(* Logix 5000 AddOnInstructionDefinition export Banner_R95C_4B4UI_Param_v4; software revision 36.00 *)

TYPE Banner_Direct1_v4 :
STRUCT
   Reserved : INT;
   Master_Cycle_Time : INT;
   Min_Cycle_Time : INT;
   M_Sequence_Capability : INT;
   IO_Link_Version_ID : INT;
   Process_Data_Input_Length : INT;
   Process_Data_Output_Length : INT;
   Vendor_ID1 : INT;
   Vendor_ID2 : INT;
   Device_ID1 : INT;
   Device_ID2 : INT;
   Device_ID3 : INT;
END_STRUCT
END_TYPE

TYPE Banner_IOL_Port_v4 :   // UDT that has all of the data items necessary to communicate with a specific Port on a IO-Link Master
STRUCT
   Port_Controlled : INT;   // Each bit represents a port on an IO-Link Master. Set to 1 to tell AOI to control that port.
   Port_Activate : INT;   // Each bit represents a port on an IO-Link Master. When ON that port will process any commands in queue.
   Port_Read : INT;   // Each bit represents a port on an IO-Link Master. Used to determine when device AOI has requested a Read command.
   Port_Write : INT;   // Each bit represents a port on an IO-Link Master. Used to determine when device AOI has requested a Write command.
   Port_RW_Complete : INT;   // Each bit represents a port on an IO-Link Master. Tells device AOI that Read or Write request has been completed.
   Port_Device_Read : INT;
   Data_Transfer : SINT[190];   // Array to transfer data from IO-Master to device AOIs.
END_STRUCT
END_TYPE

TYPE Banner_Locks_v4 :
STRUCT
   Parameter_Access_Lock : SINT;   // Write access to all parameters is prohibited while value is 1. Only this parameter can be adjusted when value is 1.
   Data_Storage_Lock : SINT;   // Automatic data storage is disabled when this value is equal to 1. Read access is not affected.
   Local_Parameterization_Lock : SINT;   // Parameterization via local control elements on device is disabled.
   Local_User_Interface_Lock : SINT;   // Operation of local user interface is disabled.
END_STRUCT
END_TYPE

TYPE Banner_R95C_4B4UI_IO_Metrics_v4 :
STRUCT
   Port_Discrete2_Totalizer : DINT;
   Port_Discrete2_Events_Per_Minute : DINT;
   Port_Discrete2_Duration : DINT;
   Port_Discrete2_Count : DINT;
   Port_Discrete1_Totalizer : DINT;
   Port_Discrete1_Events_Per_Minute : DINT;
   Port_Discrete1_Duration : DINT;
   Port_Discrete1_Count : DINT;
END_STRUCT
END_TYPE

TYPE Banner_R95C_4B4UI_MDC_v4 :   // MDC Descriptor parameters for Smart Sensor Profile 2nd edition.
STRUCT
   Lower_Limit : DINT;
   Upper_Limit : DINT;
   Unit : INT;   // 1209 = A, 1240 = V
   Scale : SINT;
END_STRUCT
END_TYPE

TYPE Banner_R95C_4B4UI_Metrics_v4 :
STRUCT
   Port4 : Banner_R95C_4B4UI_IO_Metrics_v4;
   Port3 : Banner_R95C_4B4UI_IO_Metrics_v4;
   Port2 : Banner_R95C_4B4UI_IO_Metrics_v4;
   Port1 : Banner_R95C_4B4UI_IO_Metrics_v4;
END_STRUCT
END_TYPE

TYPE Banner_R95C_4B4UI_Port_Config_v4 :
STRUCT
   D2 : Banner_R95C_4B4UI_Port_Discrete_v4;   // Discrete 2
   D1 : Banner_R95C_4B4UI_Port_Discrete_v4;   // Discrete 1
END_STRUCT
END_TYPE

TYPE Banner_R95C_4B4UI_Port_Discrete_v4 :
STRUCT
   PFM_Far_Freq : DINT;   // 100 to 600.
   PFM_Near_Freq : DINT;   // 100 to 600.
   Mirroring_Inversion : SINT;   // 0 = Not Inverted, 1 = Inverted.
   Mirroring_Channel_Selection : SINT;   // 0 = Discrete 1, 1 = Discrete 2.
   Mirroring_Port_Selection : SINT;   // 0 = Port1, 1 = Port2, 2 = Port3, 3 = Prot4, 4 = Prot5, 5 = Port6, 6 = Port7, 7 = Port8.
   Mirroring_Enable : SINT;   // 0 = Disabled, 1 = Enabled.
   Delay_Timer2 : DINT;
   Delay_Timer1 : DINT;
   Delay_Mode : SINT;   // 0=Disabled,1=On Off Delay, 2=On OneShot, 3=Off OneShot, 4=On Pulse Stretcher, 5=Off Pulse Stretcher, 6=Totalizer, 7=Retriggerable On OneShot, 8=Retriggerable Off OneShot.
   IO : SINT;   // 0=NPN, 1=PNP
END_STRUCT
END_TYPE

TYPE Banner_R95C_4B4UI_Port_Mirroring_v4 :
STRUCT
   Output_Enable : SINT;   // 0 = Disabled, 1 = Enabled. Enable mirroring over output analog channel.
   Port_Selection : SINT;   // 0 = Port 5, 1 = Port 6, 2 = Port 7, 3 = Port 8. Input port to mirror over output analog channel.
END_STRUCT
END_TYPE

TYPE Banner_R95C_4B4UI_POVR1_v4 :
STRUCT
   PDO8_OVD : SINT;   // 0 = Hold, 1 = Low, 2 = High. Value sensor will output when PDO value is not within allowable range.
   PDO7_OVD : SINT;   // 0 = Hold, 1 = Low, 2 = High. Value sensor will output when PDO value is not within allowable range.
   PDO6_OVD : SINT;   // 0 = Hold, 1 = Low, 2 = High. Value sensor will output when PDO value is not within allowable range.
   PDO5_OVD : SINT;   // 0 = Hold, 1 = Low, 2 = High. Value sensor will output when PDO value is not within allowable range.
END_STRUCT
END_TYPE

TYPE Banner_R95C_4B4UI_RD_v4 :   // UDT that stores the Read Data for a R95C-4B4UI-KQ.
STRUCT
   Direct1 : Banner_Direct1_v4;
   Combined_Vendor_ID : DINT;   // IO-Link Vendor ID
   Combined_Device_ID : DINT;   // IO-Link Device ID
   Serial_Number : STRING;
   All_Time_Run_Time : DINT;
   IO_Metrics_1_to_4 : Banner_R95C_4B4UI_Metrics_v4;
   MDC_5_to_8 : Banner_R95C_4B4UI_MDC_v4[4];
END_STRUCT
END_TYPE

TYPE Banner_R95C_4B4UI_Setpoints_v4 :   // The Channel setpoints for a R95C-4B4UI-KQ.
STRUCT
   Current_Hysteresis : DINT;   // Hysteresis value for the current switchpont.
   Current_SP2 : DINT;   // Upper limit setpoint.
   Current_SP1 : DINT;   // Lower limit setpoint.
   Voltage_Hysteresis : DINT;   // Hysteresis value for the voltage switchpont.
   Voltage_SP2 : DINT;   // Upper limit setpoint.
   Voltage_SP1 : DINT;   // Lower limit setpoint.
END_STRUCT
END_TYPE

TYPE Banner_R95C_4B4UI_SMR_Port_v4 :
STRUCT
   P4_D2_Reset_Count : DINT;   // Port 4 Discrete 2. Value that Counter is set to when a Reset Metrics operation is activated.
   P4_D1_Reset_Count : DINT;   // Port 4 Discrete 1. Value that Counter is set to when a Reset Metrics operation is activated.
   P3_D2_Reset_Count : DINT;   // Port 3 Discrete 2. Value that Counter is set to when a Reset Metrics operation is activated.
   P3_D1_Reset_Count : DINT;   // Port 3 Discrete 1. Value that Counter is set to when a Reset Metrics operation is activated.
   P2_D2_Reset_Count : DINT;   // Port 2 Discrete 2. Value that Counter is set to when a Reset Metrics operation is activated.
   P2_D1_Reset_Count : DINT;   // Port 2 Discrete 1. Value that Counter is set to when a Reset Metrics operation is activated.
   P1_D2_Reset_Count : DINT;   // Port 1 Discrete 2. Value that Counter is set to when a Reset Metrics operation is activated.
   P1_D1_Reset_Count : DINT;   // Port 1 Discrete 1. Value that Counter is set to when a Reset Metrics operation is activated.
   Reserved1 : DINT;
   P1_Discrete1 : SINT;   // 0 = Normal setting, 1 = Reset metrics.
   P1_Discrete2 : SINT;   // 0 = Normal setting, 1 = Reset metrics.
   P2_Discrete1 : SINT;   // 0 = Normal setting, 1 = Reset metrics.
   P2_Discrete2 : SINT;   // 0 = Normal setting, 1 = Reset metrics.
   P3_Discrete1 : SINT;   // 0 = Normal setting, 1 = Reset metrics.
   P3_Discrete2 : SINT;   // 0 = Normal setting, 1 = Reset metrics.
   P4_Discrete1 : SINT;   // 0 = Normal setting, 1 = Reset metrics.
   P4_Discrete2 : SINT;   // 0 = Normal setting, 1 = Reset metrics.
END_STRUCT
END_TYPE

TYPE Banner_R95C_4B4UI_v4 :   // All of the parameters for a R95C-4B4UI-KQ.
STRUCT
   Initial_Global_Read : BOOL;   // Determines if all of the IO-Link data has been read into the PLC yet
   Command : INT;   // Value placed in here will activate a read or write to a specifc IO-Link Index
   Read : Banner_R95C_4B4UI_RD_v4;   // Read Only Data
   Write : Banner_R95C_4B4UI_WD_v4;   // Write Data
   Archive : Banner_R95C_4B4UI_WD_v4;   // Archive of the Write Data
   Reset : BOOL;   // Resets AOI. This will force a complete parameter read of the sensor.
END_STRUCT
END_TYPE

TYPE Banner_R95C_4B4UI_VSC_Analog_v4 :
STRUCT
   P8_Analog_Out_Mode : SINT;   // 0 = Voltage, 1 = Current.
   P7_Analog_Out_Mode : SINT;   // 0 = Voltage, 1 = Current.
   P6_Analog_Out_Mode : SINT;   // 0 = Voltage, 1 = Current.
   P5_Analog_Out_Mode : SINT;   // 0 = Voltage, 1 = Current.
   P8_Mode_Analog_In : SINT;   // 0 = Voltage, 1 = Current.
   P7_Mode_Analog_In : SINT;   // 0 = Voltage, 1 = Current.
   P6_Mode_Analog_In : SINT;   // 0 = Voltage, 1 = Current.
   P5_Mode_Analog_In : SINT;   // 0 = Voltage, 1 = Current.
END_STRUCT
END_TYPE

TYPE Banner_R95C_4B4UI_VSC_Measure_v4 :
STRUCT
   Channel_Selection : SINT;   // 0 = Discrete 1, 1 = Discrete 2
   Port_Selection : SINT;   // 0 = Port 1, 1 = Port 2, 2 = Port 3, 3 = Port 4
   Metric_Selection : SINT;   // 0 = Disabled, 1 = Count, 2 = Duration, 3 = Events Per Minute.
END_STRUCT
END_TYPE

TYPE Banner_R95C_4B4UI_VSC_v4 :   // Vendor Specific Configuration data elements for a R95C-4B4UI-KQ.
STRUCT
   Analog : Banner_R95C_4B4UI_VSC_Analog_v4;
   IOL_Filter_Time : INT;   // Timer to average IOL process data measurement between updates.
   POVR : Banner_R95C_4B4UI_POVR1_v4;
   Measure4 : Banner_R95C_4B4UI_VSC_Measure_v4;
   Measure3 : Banner_R95C_4B4UI_VSC_Measure_v4;
   Measure2 : Banner_R95C_4B4UI_VSC_Measure_v4;
   Measure1 : Banner_R95C_4B4UI_VSC_Measure_v4;
   PDI_Config : SINT;   // 0 = Analog Value, 1 = Digital Measuring Sensor.
END_STRUCT
END_TYPE

TYPE Banner_R95C_4B4UI_WD_v4 :   // UDT that stores the Write Data for a R95C-4B4UI-KQ.
STRUCT
   System_Command : INT;   // See IODD file for list of commands that can be activated via the System Command interface
   Locks : Banner_Locks_v4;
   PM : Banner_R95C_4B4UI_Port_Mirroring_v4[4];   // Port Mirroring. 0 = 5, 1, = 6, 2 = 7, 3 = 8.
   Resettable_Run_Time : DINT;   // Read/Write time counter in hours.
   VSC : Banner_R95C_4B4UI_VSC_v4;
   All_Time_Run_Time_Event_Time : DINT;   // Event indicating the corresponding configured running time has elapsed.
   Resettable_Run_Time_Event_TIme : DINT;   // Running time when an event will be raised indicating that service is required.
   SMR : Banner_R95C_4B4UI_SMR_Port_v4;   // Selectable Metric Reset
   Port : Banner_R95C_4B4UI_Port_Config_v4[5];   // Port Configuration
   Setpoints_5_to_8 : Banner_R95C_4B4UI_Setpoints_v4[4];   // 0 = 5, 1, = 6, 2 = 7, 3 = 8.
END_STRUCT
END_TYPE

ADD_ON_INSTRUCTION Banner_R95C_4B4UI_Param_v4   (* revision 4.0, vendor Banner Engineering *)
// AOI to read and write parameter data to an IO-Link R95C-4B4UI-KQ.
VAR_IN_OUT
   R95C : Banner_R95C_4B4UI_v4; {required}
   Port_Data : Banner_IOL_Port_v4; {required}
END_VAR
VAR_INPUT
   Port : INT; {required}   // Port Number that device is plugged into.
END_VAR
VAR
   Local_Control : DINT; {access None}
   Global_Read_Command_Value : INT; {access None}
   Global_Write_Command_Value : INT; {access None}
   Command_Being_Processed : BOOL; {access None}
   Update_Archive : BOOL; {access None}
   Index_Write_Inprocess : DINT; {access None}
   Index_Write_Control : DINT; {access None}
   Inprocess_Index : DINT; {access None}
   Index1 : DINT; {access None}
   Index2 : DINT; {access None}
   Index3 : DINT; {access None}
   Index_Segment_Read : DINT; {access None}
   Index_PM : DINT; {access None}
   Index4 : DINT; {access None}
END_VAR

ROUTINE Logic   (* ladder *)
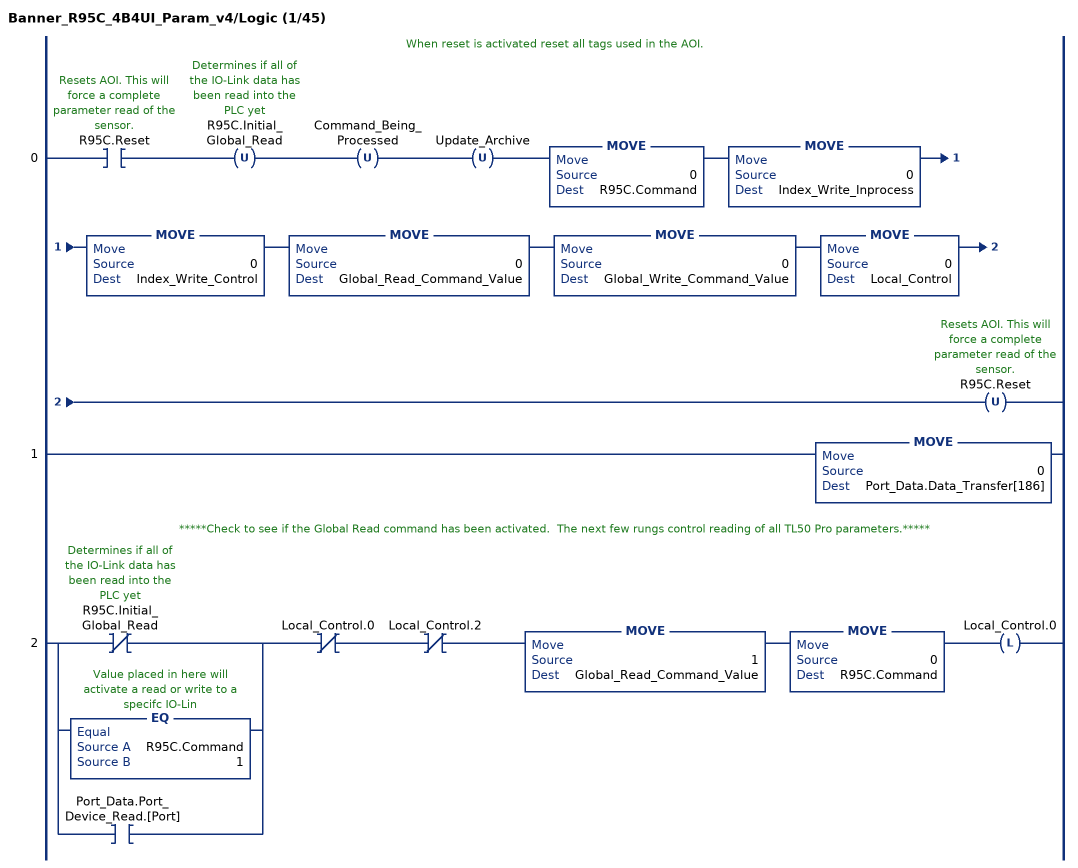
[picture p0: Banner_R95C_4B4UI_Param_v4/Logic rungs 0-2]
   // When reset is activated reset all tags used in the AOI.
   0: XIC(R95C.Reset)OTU(R95C.Initial_Global_Read)OTU(Command_Being_Processed)OTU(Update_Archive)MOVE(0,R95C.Command)MOVE(0,Index_Write_Inprocess)MOVE(0,Index_Write_Control)MOVE(0,Global_Read_Command_Value)MOVE(0,Global_Write_Command_Value)MOVE(0,Local_Control)OTU(R95C.Reset);
   1: MOVE(0,Port_Data.Data_Transfer[186]);
   // *****Check to see if the Global Read command has been activated.  The next few rungs control reading of all TL50 Pro parameters.*****
   2: [XIO(R95C.Initial_Global_Read) ,EQ(R95C.Command,1) ,XIC(Port_Data.Port_Device_Read.[Port]) ]XIO(Local_Control.0)XIO(Local_Control.2)MOVE(1,Global_Read_Command_Value)MOVE(0,R95C.Command)OTL(Local_Control.0);
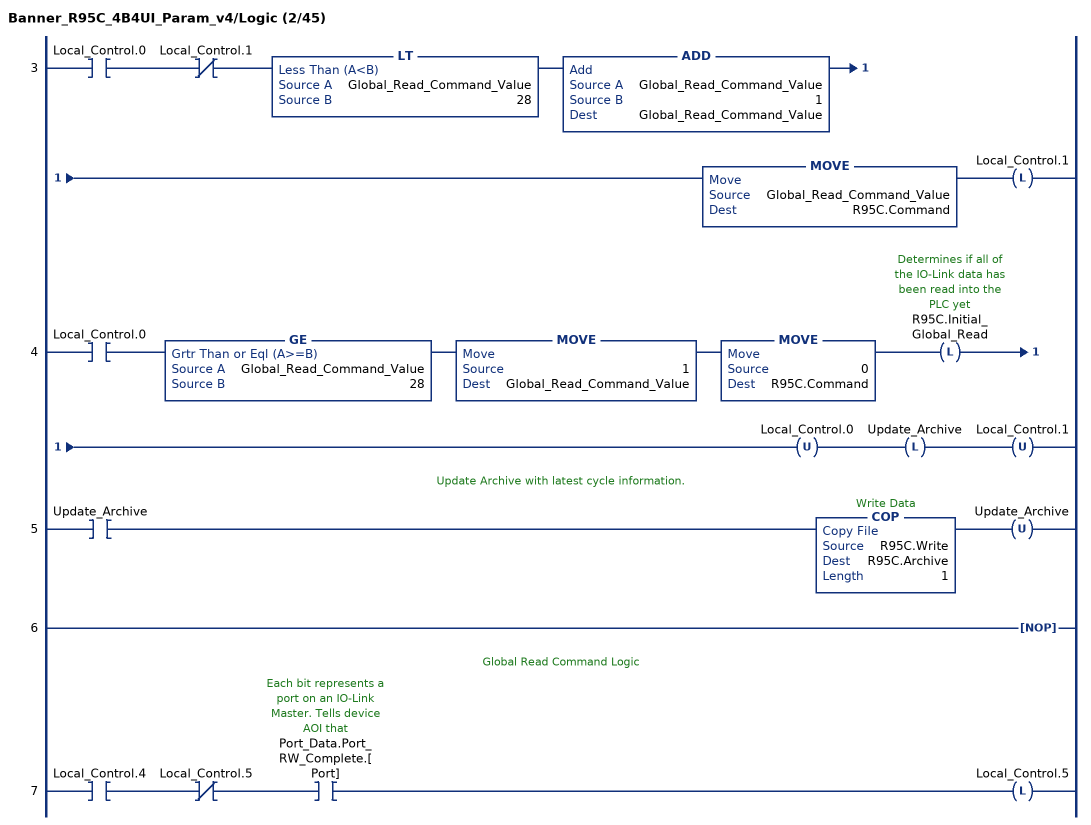
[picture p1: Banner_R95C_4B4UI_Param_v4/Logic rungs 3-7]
   3: XIC(Local_Control.0)XIO(Local_Control.1)LT(Global_Read_Command_Value,28)ADD(Global_Read_Command_Value,1,Global_Read_Command_Value)MOVE(Global_Read_Command_Value,R95C.Command)OTL(Local_Control.1);
   4: XIC(Local_Control.0)GE(Global_Read_Command_Value,28)MOVE(1,Global_Read_Command_Value)MOVE(0,R95C.Command)OTL(R95C.Initial_Global_Read)OTU(Local_Control.0)OTL(Update_Archive)OTU(Local_Control.1);
   // Update Archive with latest cycle information.
   5: XIC(Update_Archive)COP(R95C.Write,R95C.Archive,1)OTU(Update_Archive);
   6: NOP();
   // Global Read Command Logic
   7: XIC(Local_Control.4)XIO(Local_Control.5)XIC(Port_Data.Port_RW_Complete.[Port])OTL(Local_Control.5);
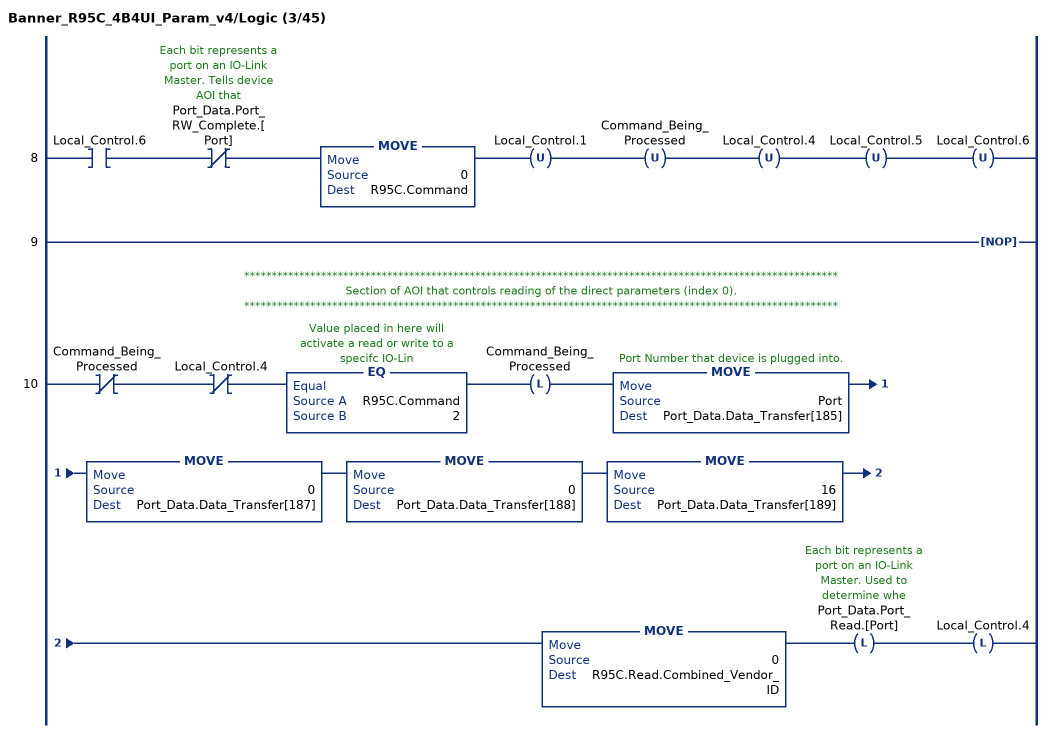
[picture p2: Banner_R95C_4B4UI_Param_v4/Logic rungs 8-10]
   8: XIC(Local_Control.6)XIO(Port_Data.Port_RW_Complete.[Port])MOVE(0,R95C.Command)OTU(Local_Control.1)OTU(Command_Being_Processed)OTU(Local_Control.4)OTU(Local_Control.5)OTU(Local_Control.6);
   9: NOP();
   // ************************************************************************************************************
   // Section of AOI that controls reading of the direct parameters (index 0).
   // ************************************************************************************************************
   10: XIO(Command_Being_Processed)XIO(Local_Control.4)EQ(R95C.Command,2)OTL(Command_Being_Processed)MOVE(Port,Port_Data.Data_Transfer[185])MOVE(0,Port_Data.Data_Transfer[187])MOVE(0,Port_Data.Data_Transfer[188])MOVE(16,Port_Data.Data_Transfer[189])MOVE(0,R95C.Read.Combined_Vendor_ID)OTL(Port_Data.Port_Read.[Port])OTL(Local_Control.4);
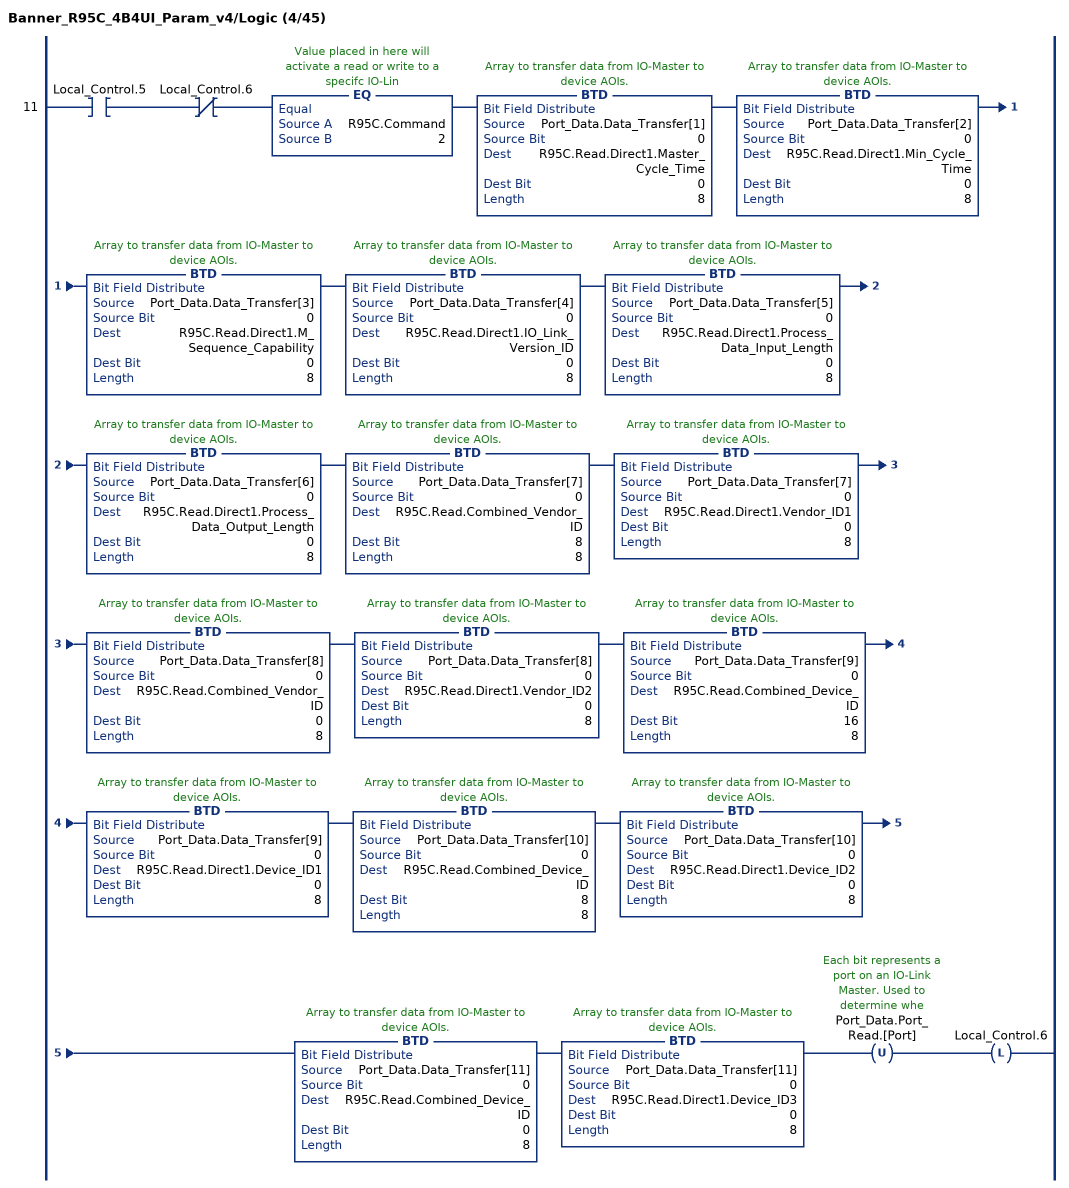
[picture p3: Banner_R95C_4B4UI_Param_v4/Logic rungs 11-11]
   11: XIC(Local_Control.5)XIO(Local_Control.6)EQ(R95C.Command,2)BTD(Port_Data.Data_Transfer[1],0,R95C.Read.Direct1.Master_Cycle_Time,0,8)BTD(Port_Data.Data_Transfer[2],0,R95C.Read.Direct1.Min_Cycle_Time,0,8)BTD(Port_Data.Data_Transfer[3],0,R95C.Read.Direct1.M_Sequence_Capability,0,8)BTD(Port_Data.Data_Transfer[4],0,R95C.Read.Direct1.IO_Link_Version_ID,0,8)BTD(Port_Data.Data_Transfer[5],0,R95C.Read.Direct1.Process_Data_Input_Length,0,8)BTD(Port_Data.Data_Transfer[6],0,R95C.Read.Direct1.Process_Data_Output_Length,0,8)BTD(Port_Data.Data_Transfer[7],0,R95C.Read.Combined_Vendor_ID,8,8)BTD(Port_Data.Data_Transfer[7],0,R95C.Read.Direct1.Vendor_ID1,0,8)BTD(Port_Data.Data_Transfer[8],0,R95C.Read.Combined_Vendor_ID,0,8)BTD(Port_Data.Data_Transfer[8],0,R95C.Read.Direct1.Vendor_ID2,0,8)BTD(Port_Data.Data_Transfer[9],0,R95C.Read.Combined_Device_ID,16,8)BTD(Port_Data.Data_Transfer[9],0,R95C.Read.Direct1.Device_ID1,0,8)BTD(Port_Data.Data_Transfer[10],0,R95C.Read.Combined_Device_ID,8,8)BTD(Port_Data.Data_Transfer[10],0,R95C.Read.Direct1.Device_ID2,0,8)BTD(Port_Data.Data_Transfer[11],0,R95C.Read.Combined_Device_ID,0,8)BTD(Port_Data.Data_Transfer[11],0,R95C.Read.Direct1.Device_ID3,0,8)OTU(Port_Data.Port_Read.[Port])OTL(Local_Control.6);
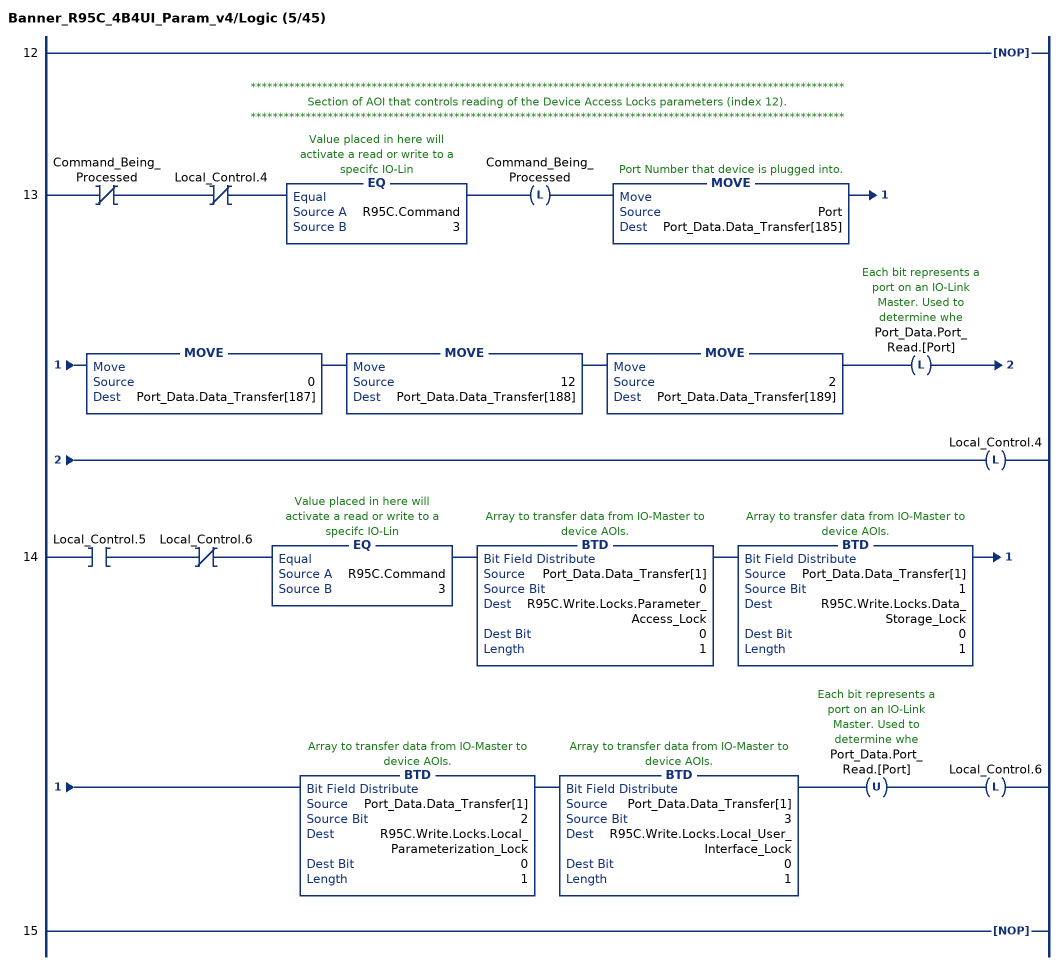
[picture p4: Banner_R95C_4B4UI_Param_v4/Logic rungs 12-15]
   12: NOP();
   // ************************************************************************************************************
   // Section of AOI that controls reading of the Device Access Locks parameters (index 12).
   // ************************************************************************************************************
   13: XIO(Command_Being_Processed)XIO(Local_Control.4)EQ(R95C.Command,3)OTL(Command_Being_Processed)MOVE(Port,Port_Data.Data_Transfer[185])MOVE(0,Port_Data.Data_Transfer[187])MOVE(12,Port_Data.Data_Transfer[188])MOVE(2,Port_Data.Data_Transfer[189])OTL(Port_Data.Port_Read.[Port])OTL(Local_Control.4);
   14: XIC(Local_Control.5)XIO(Local_Control.6)EQ(R95C.Command,3)BTD(Port_Data.Data_Transfer[1],0,R95C.Write.Locks.Parameter_Access_Lock,0,1)BTD(Port_Data.Data_Transfer[1],1,R95C.Write.Locks.Data_Storage_Lock,0,1)BTD(Port_Data.Data_Transfer[1],2,R95C.Write.Locks.Local_Parameterization_Lock,0,1)BTD(Port_Data.Data_Transfer[1],3,R95C.Write.Locks.Local_User_Interface_Lock,0,1)OTU(Port_Data.Port_Read.[Port])OTL(Local_Control.6);
   15: NOP();
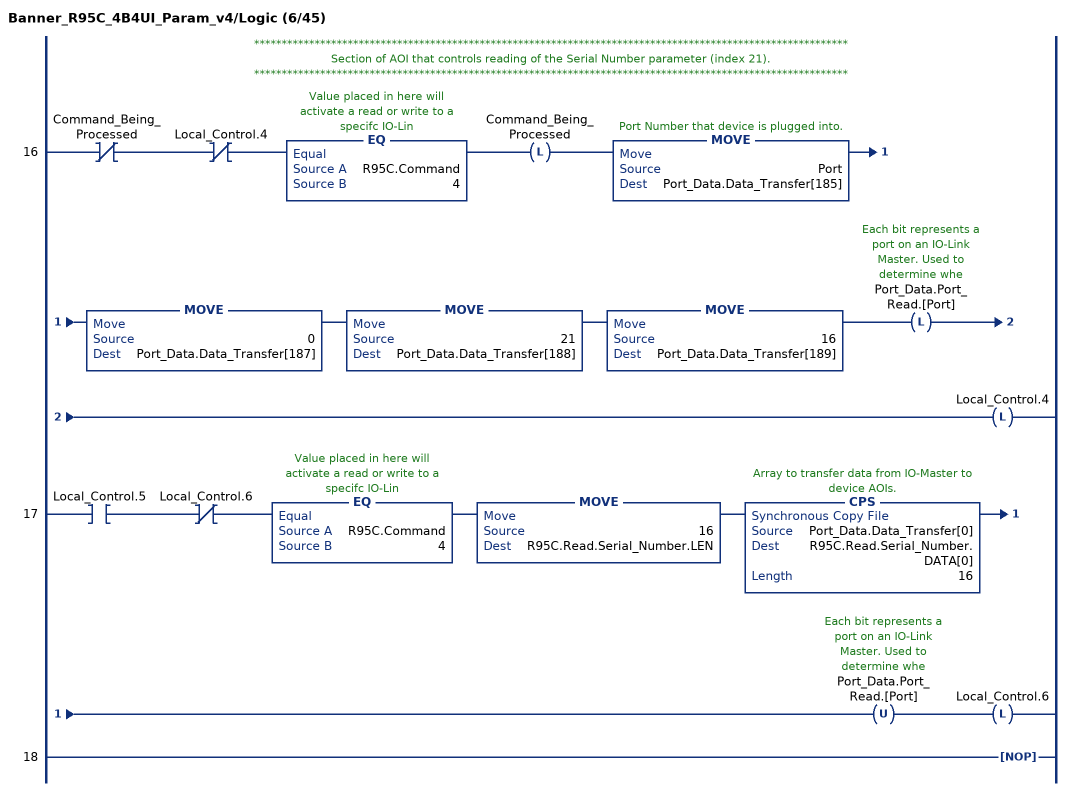
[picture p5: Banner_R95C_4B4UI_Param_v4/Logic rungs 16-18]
   // ************************************************************************************************************
   // Section of AOI that controls reading of the Serial Number parameter (index 21).
   // ************************************************************************************************************
   16: XIO(Command_Being_Processed)XIO(Local_Control.4)EQ(R95C.Command,4)OTL(Command_Being_Processed)MOVE(Port,Port_Data.Data_Transfer[185])MOVE(0,Port_Data.Data_Transfer[187])MOVE(21,Port_Data.Data_Transfer[188])MOVE(16,Port_Data.Data_Transfer[189])OTL(Port_Data.Port_Read.[Port])OTL(Local_Control.4);
   17: XIC(Local_Control.5)XIO(Local_Control.6)EQ(R95C.Command,4)MOVE(16,R95C.Read.Serial_Number.LEN)CPS(Port_Data.Data_Transfer[0],R95C.Read.Serial_Number.DATA[0],16)OTU(Port_Data.Port_Read.[Port])OTL(Local_Control.6);
   18: NOP();
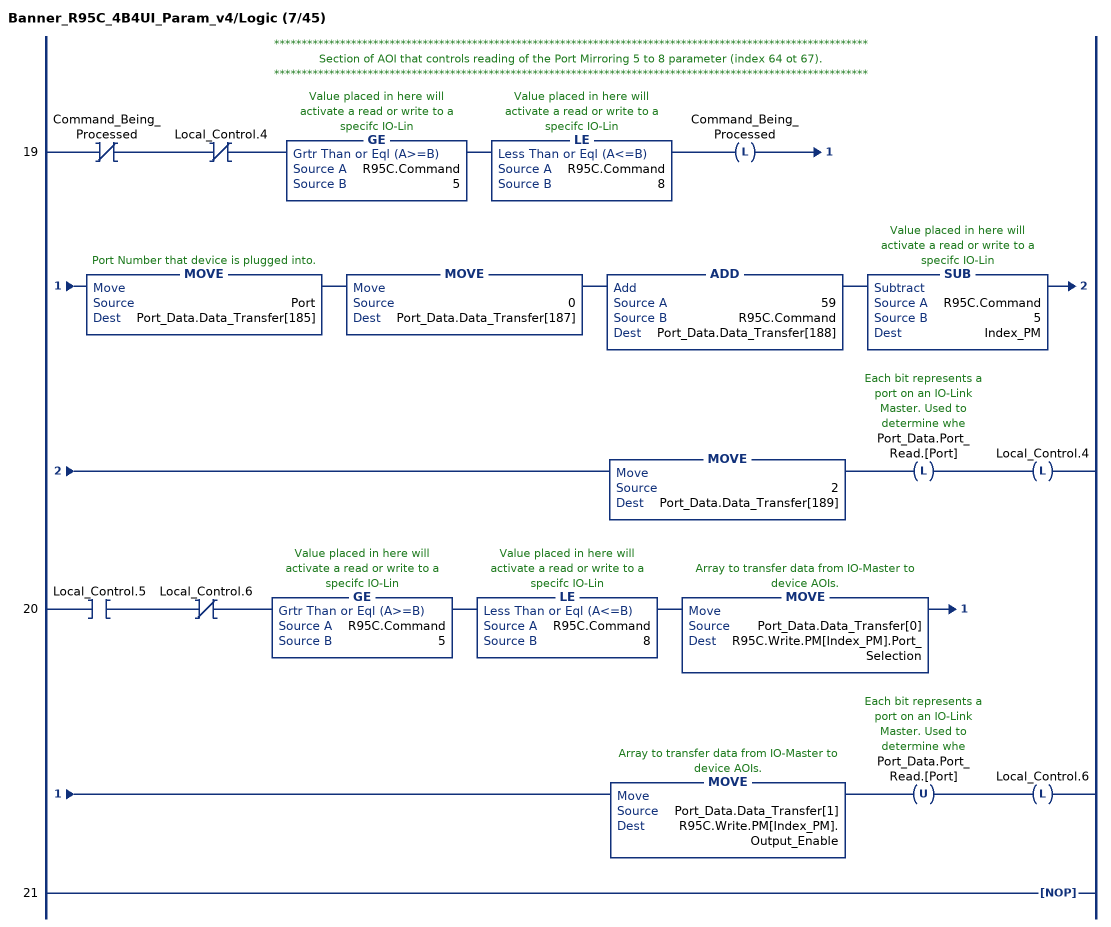
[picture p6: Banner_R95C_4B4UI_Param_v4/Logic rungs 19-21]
   // ************************************************************************************************************
   // Section of AOI that controls reading of the Port Mirroring 5 to 8 parameter (index 64 ot 67).
   // ************************************************************************************************************
   19: XIO(Command_Being_Processed)XIO(Local_Control.4)GE(R95C.Command,5)LE(R95C.Command,8)OTL(Command_Being_Processed)MOVE(Port,Port_Data.Data_Transfer[185])MOVE(0,Port_Data.Data_Transfer[187])ADD(59,R95C.Command,Port_Data.Data_Transfer[188])SUB(R95C.Command,5,Index_PM)MOVE(2,Port_Data.Data_Transfer[189])OTL(Port_Data.Port_Read.[Port])OTL(Local_Control.4);
   20: XIC(Local_Control.5)XIO(Local_Control.6)GE(R95C.Command,5)LE(R95C.Command,8)MOVE(Port_Data.Data_Transfer[0],R95C.Write.PM[Index_PM].Port_Selection)MOVE(Port_Data.Data_Transfer[1],R95C.Write.PM[Index_PM].Output_Enable)OTU(Port_Data.Port_Read.[Port])OTL(Local_Control.6);
   21: NOP();
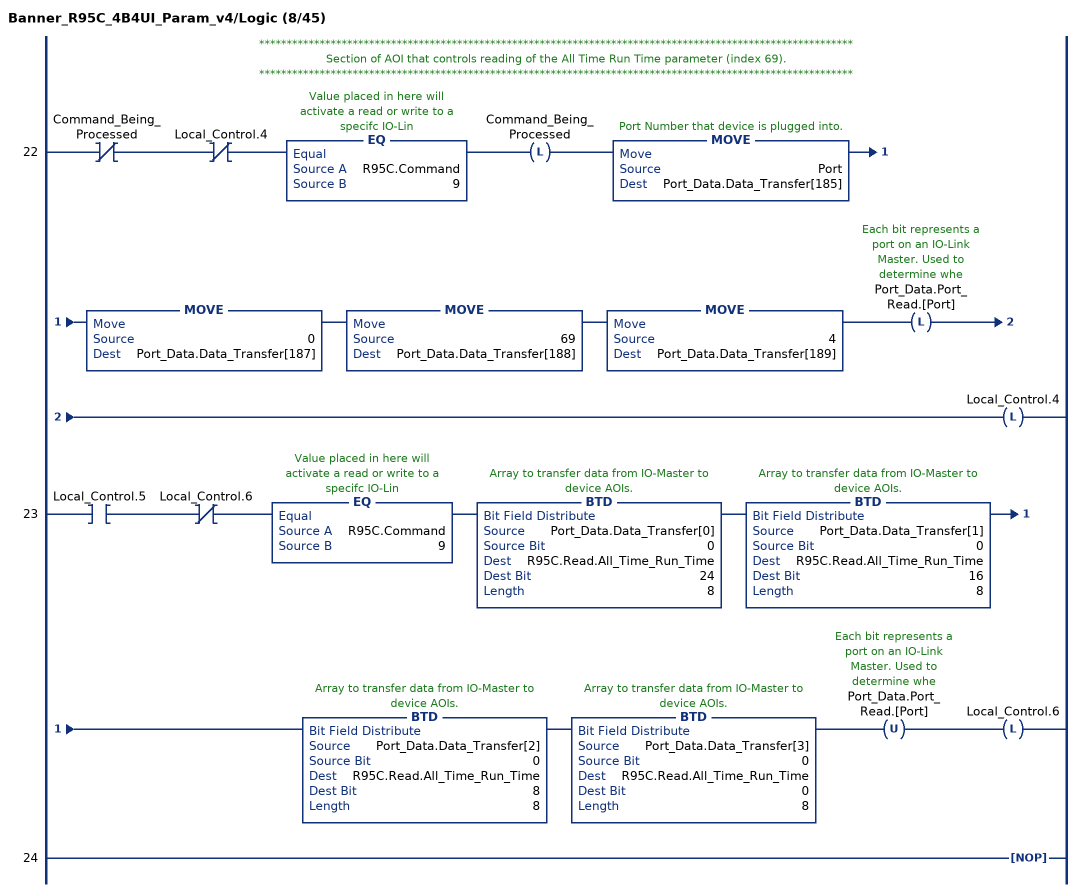
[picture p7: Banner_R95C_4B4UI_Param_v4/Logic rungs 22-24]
   // ************************************************************************************************************
   // Section of AOI that controls reading of the All Time Run Time parameter (index 69).
   // ************************************************************************************************************
   22: XIO(Command_Being_Processed)XIO(Local_Control.4)EQ(R95C.Command,9)OTL(Command_Being_Processed)MOVE(Port,Port_Data.Data_Transfer[185])MOVE(0,Port_Data.Data_Transfer[187])MOVE(69,Port_Data.Data_Transfer[188])MOVE(4,Port_Data.Data_Transfer[189])OTL(Port_Data.Port_Read.[Port])OTL(Local_Control.4);
   23: XIC(Local_Control.5)XIO(Local_Control.6)EQ(R95C.Command,9)BTD(Port_Data.Data_Transfer[0],0,R95C.Read.All_Time_Run_Time,24,8)BTD(Port_Data.Data_Transfer[1],0,R95C.Read.All_Time_Run_Time,16,8)BTD(Port_Data.Data_Transfer[2],0,R95C.Read.All_Time_Run_Time,8,8)BTD(Port_Data.Data_Transfer[3],0,R95C.Read.All_Time_Run_Time,0,8)OTU(Port_Data.Port_Read.[Port])OTL(Local_Control.6);
   24: NOP();
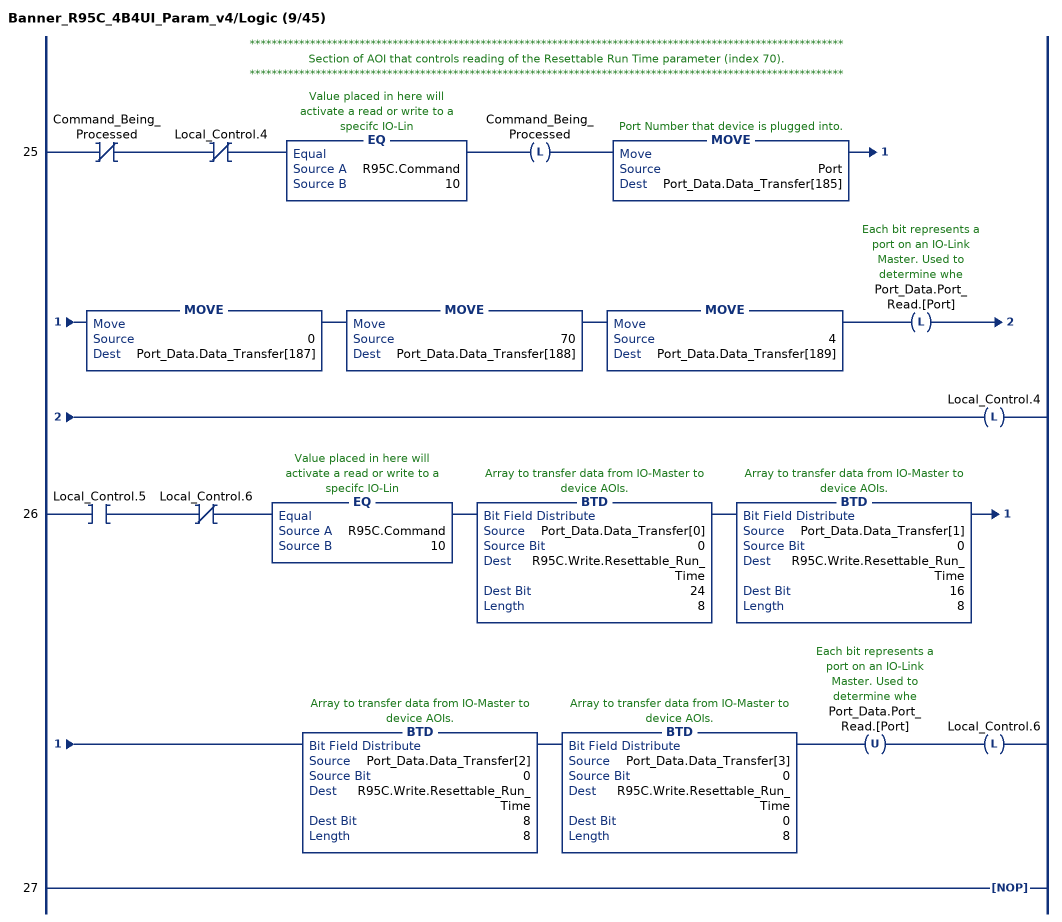
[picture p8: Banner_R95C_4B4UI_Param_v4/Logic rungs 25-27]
   // ************************************************************************************************************
   // Section of AOI that controls reading of the Resettable Run Time parameter (index 70).
   // ************************************************************************************************************
   25: XIO(Command_Being_Processed)XIO(Local_Control.4)EQ(R95C.Command,10)OTL(Command_Being_Processed)MOVE(Port,Port_Data.Data_Transfer[185])MOVE(0,Port_Data.Data_Transfer[187])MOVE(70,Port_Data.Data_Transfer[188])MOVE(4,Port_Data.Data_Transfer[189])OTL(Port_Data.Port_Read.[Port])OTL(Local_Control.4);
   26: XIC(Local_Control.5)XIO(Local_Control.6)EQ(R95C.Command,10)BTD(Port_Data.Data_Transfer[0],0,R95C.Write.Resettable_Run_Time,24,8)BTD(Port_Data.Data_Transfer[1],0,R95C.Write.Resettable_Run_Time,16,8)BTD(Port_Data.Data_Transfer[2],0,R95C.Write.Resettable_Run_Time,8,8)BTD(Port_Data.Data_Transfer[3],0,R95C.Write.Resettable_Run_Time,0,8)OTU(Port_Data.Port_Read.[Port])OTL(Local_Control.6);
   27: NOP();
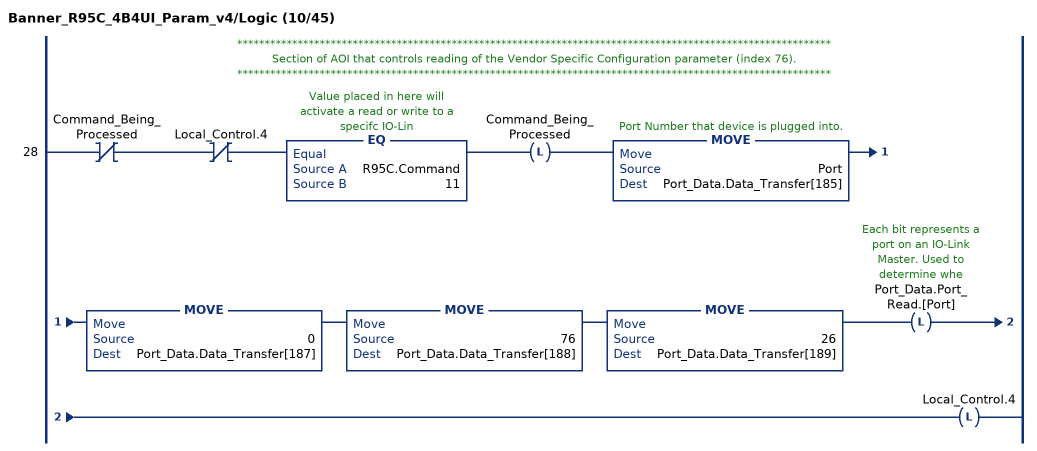
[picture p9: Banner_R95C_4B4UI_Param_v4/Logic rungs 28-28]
   // ************************************************************************************************************
   // Section of AOI that controls reading of the Vendor Specific Configuration parameter (index 76).
   // ************************************************************************************************************
   28: XIO(Command_Being_Processed)XIO(Local_Control.4)EQ(R95C.Command,11)OTL(Command_Being_Processed)MOVE(Port,Port_Data.Data_Transfer[185])MOVE(0,Port_Data.Data_Transfer[187])MOVE(76,Port_Data.Data_Transfer[188])MOVE(26,Port_Data.Data_Transfer[189])OTL(Port_Data.Port_Read.[Port])OTL(Local_Control.4);
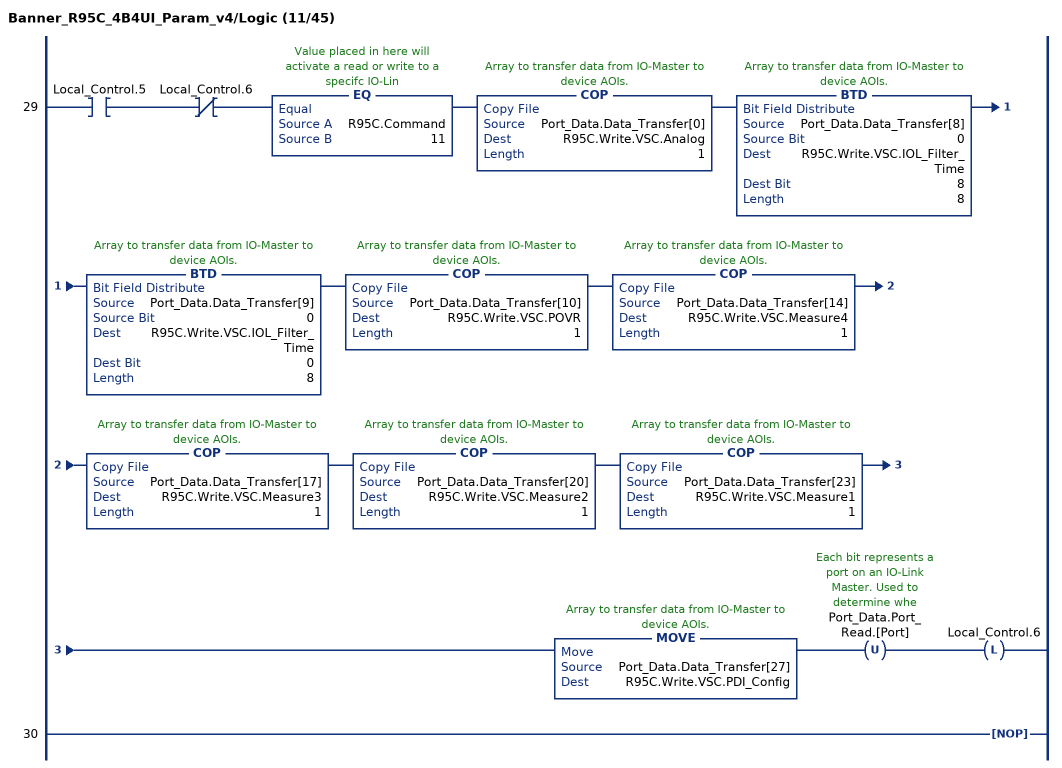
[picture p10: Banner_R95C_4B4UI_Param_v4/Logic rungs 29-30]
   29: XIC(Local_Control.5)XIO(Local_Control.6)EQ(R95C.Command,11)COP(Port_Data.Data_Transfer[0],R95C.Write.VSC.Analog,1)BTD(Port_Data.Data_Transfer[8],0,R95C.Write.VSC.IOL_Filter_Time,8,8)BTD(Port_Data.Data_Transfer[9],0,R95C.Write.VSC.IOL_Filter_Time,0,8)COP(Port_Data.Data_Transfer[10],R95C.Write.VSC.POVR,1)COP(Port_Data.Data_Transfer[14],R95C.Write.VSC.Measure4,1)COP(Port_Data.Data_Transfer[17],R95C.Write.VSC.Measure3,1)COP(Port_Data.Data_Transfer[20],R95C.Write.VSC.Measure2,1)COP(Port_Data.Data_Transfer[23],R95C.Write.VSC.Measure1,1)MOVE(Port_Data.Data_Transfer[27],R95C.Write.VSC.PDI_Config)OTU(Port_Data.Port_Read.[Port])OTL(Local_Control.6);
   30: NOP();
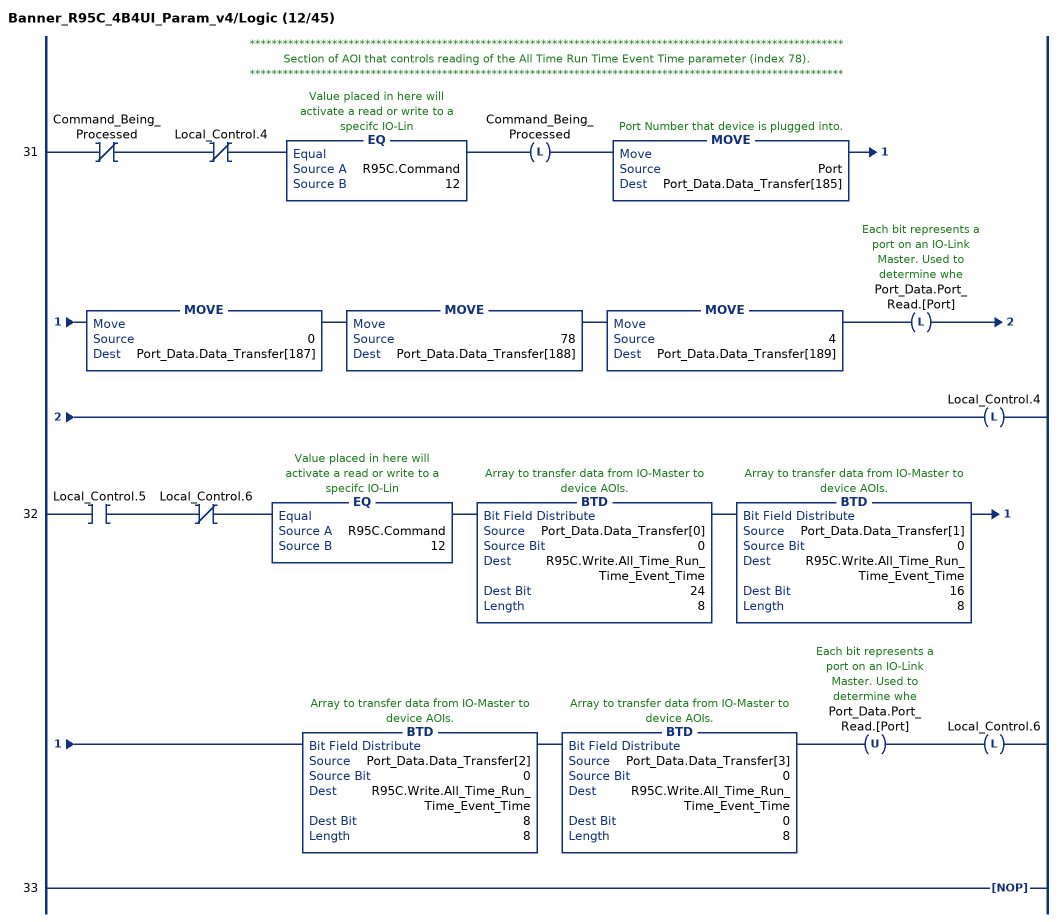
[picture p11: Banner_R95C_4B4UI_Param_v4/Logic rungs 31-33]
   // ************************************************************************************************************
   // Section of AOI that controls reading of the All Time Run Time Event Time parameter (index 78).
   // ************************************************************************************************************
   31: XIO(Command_Being_Processed)XIO(Local_Control.4)EQ(R95C.Command,12)OTL(Command_Being_Processed)MOVE(Port,Port_Data.Data_Transfer[185])MOVE(0,Port_Data.Data_Transfer[187])MOVE(78,Port_Data.Data_Transfer[188])MOVE(4,Port_Data.Data_Transfer[189])OTL(Port_Data.Port_Read.[Port])OTL(Local_Control.4);
   32: XIC(Local_Control.5)XIO(Local_Control.6)EQ(R95C.Command,12)BTD(Port_Data.Data_Transfer[0],0,R95C.Write.All_Time_Run_Time_Event_Time,24,8)BTD(Port_Data.Data_Transfer[1],0,R95C.Write.All_Time_Run_Time_Event_Time,16,8)BTD(Port_Data.Data_Transfer[2],0,R95C.Write.All_Time_Run_Time_Event_Time,8,8)BTD(Port_Data.Data_Transfer[3],0,R95C.Write.All_Time_Run_Time_Event_Time,0,8)OTU(Port_Data.Port_Read.[Port])OTL(Local_Control.6);
   33: NOP();
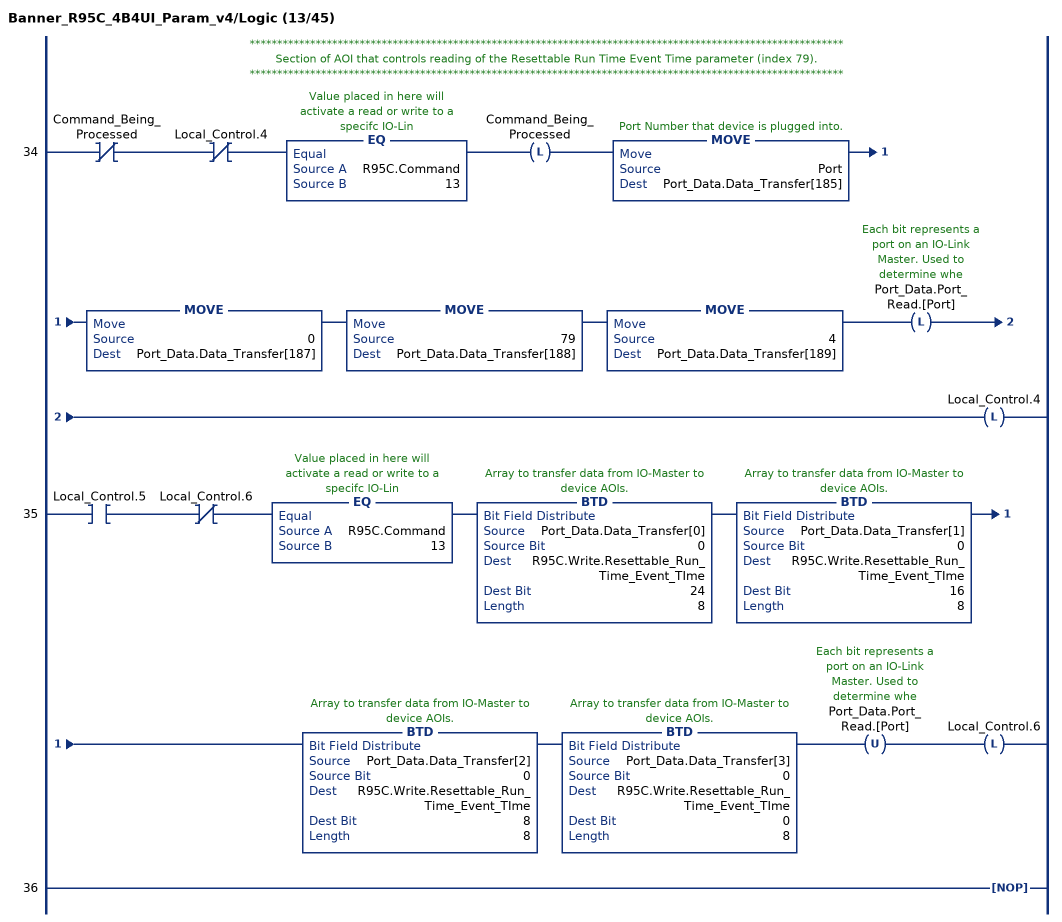
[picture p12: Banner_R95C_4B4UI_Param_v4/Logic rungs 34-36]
   // ************************************************************************************************************
   // Section of AOI that controls reading of the Resettable Run Time Event Time parameter (index 79).
   // ************************************************************************************************************
   34: XIO(Command_Being_Processed)XIO(Local_Control.4)EQ(R95C.Command,13)OTL(Command_Being_Processed)MOVE(Port,Port_Data.Data_Transfer[185])MOVE(0,Port_Data.Data_Transfer[187])MOVE(79,Port_Data.Data_Transfer[188])MOVE(4,Port_Data.Data_Transfer[189])OTL(Port_Data.Port_Read.[Port])OTL(Local_Control.4);
   35: XIC(Local_Control.5)XIO(Local_Control.6)EQ(R95C.Command,13)BTD(Port_Data.Data_Transfer[0],0,R95C.Write.Resettable_Run_Time_Event_TIme,24,8)BTD(Port_Data.Data_Transfer[1],0,R95C.Write.Resettable_Run_Time_Event_TIme,16,8)BTD(Port_Data.Data_Transfer[2],0,R95C.Write.Resettable_Run_Time_Event_TIme,8,8)BTD(Port_Data.Data_Transfer[3],0,R95C.Write.Resettable_Run_Time_Event_TIme,0,8)OTU(Port_Data.Port_Read.[Port])OTL(Local_Control.6);
   36: NOP();
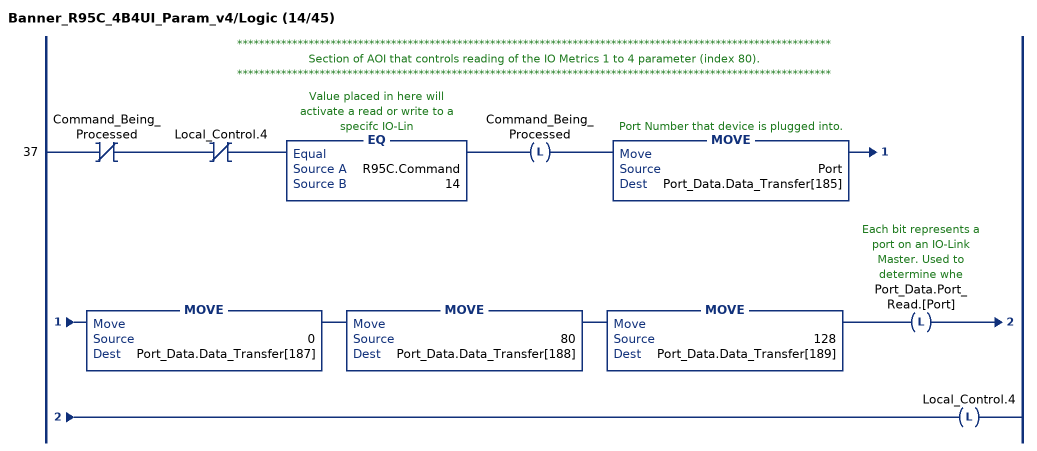
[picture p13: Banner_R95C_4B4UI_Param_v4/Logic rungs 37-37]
   // ************************************************************************************************************
   // Section of AOI that controls reading of the IO Metrics 1 to 4 parameter (index 80).
   // ************************************************************************************************************
   37: XIO(Command_Being_Processed)XIO(Local_Control.4)EQ(R95C.Command,14)OTL(Command_Being_Processed)MOVE(Port,Port_Data.Data_Transfer[185])MOVE(0,Port_Data.Data_Transfer[187])MOVE(80,Port_Data.Data_Transfer[188])MOVE(128,Port_Data.Data_Transfer[189])OTL(Port_Data.Port_Read.[Port])OTL(Local_Control.4);
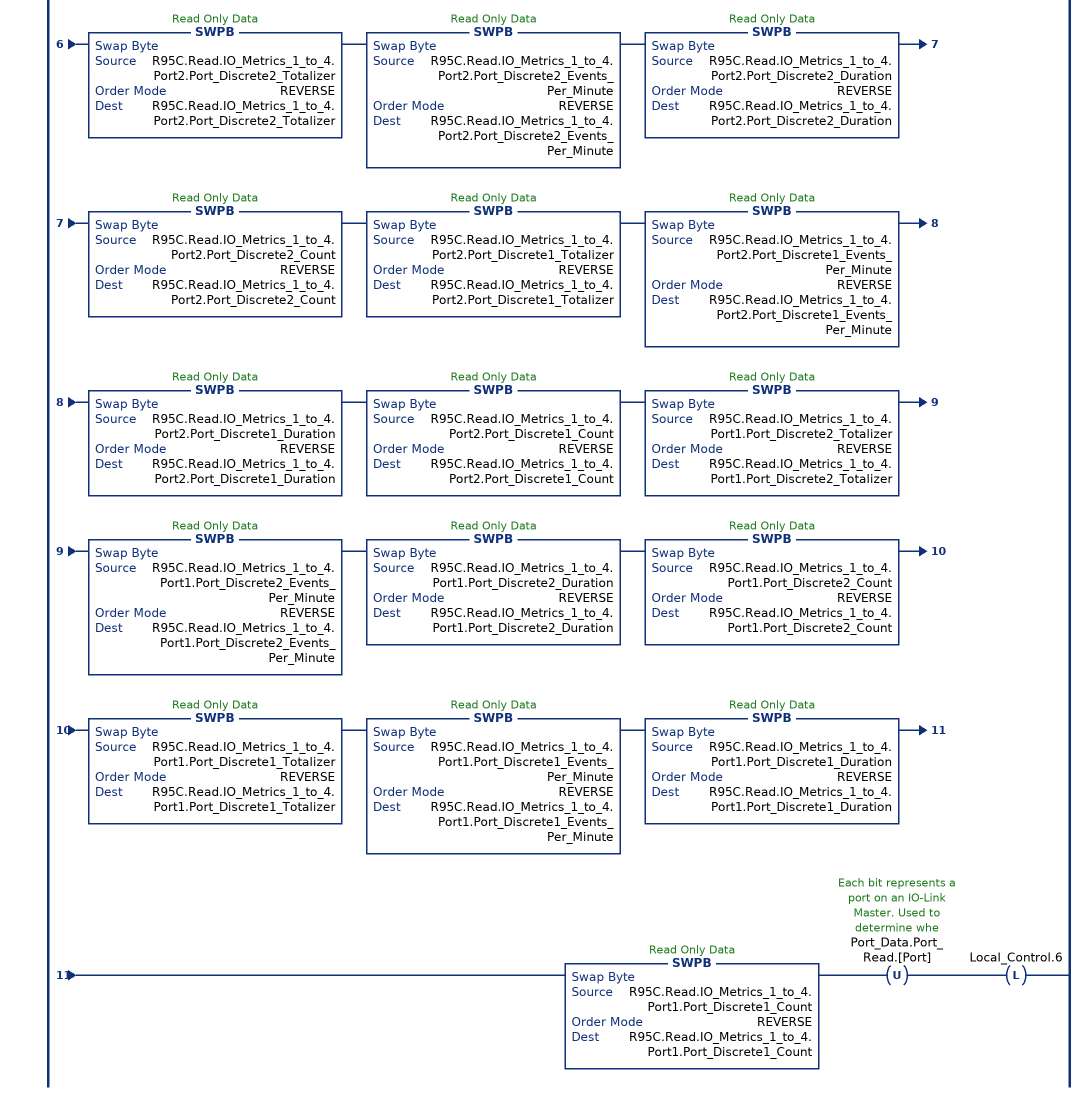
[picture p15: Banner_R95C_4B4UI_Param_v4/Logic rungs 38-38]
   38: XIC(Local_Control.5)XIO(Local_Control.6)EQ(R95C.Command,14)CPS(Port_Data.Data_Transfer[0],R95C.Read.IO_Metrics_1_to_4,1)SWPB(R95C.Read.IO_Metrics_1_to_4.Port4.Port_Discrete2_Totalizer,REVERSE,R95C.Read.IO_Metrics_1_to_4.Port4.Port_Discrete2_Totalizer)SWPB(R95C.Read.IO_Metrics_1_to_4.Port4.Port_Discrete2_Events_Per_Minute,REVERSE,R95C.Read.IO_Metrics_1_to_4.Port4.Port_Discrete2_Events_Per_Minute)SWPB(R95C.Read.IO_Metrics_1_to_4.Port4.Port_Discrete2_Duration,REVERSE,R95C.Read.IO_Metrics_1_to_4.Port4.Port_Discrete2_Duration)SWPB(R95C.Read.IO_Metrics_1_to_4.Port4.Port_Discrete2_Count,REVERSE,R95C.Read.IO_Metrics_1_to_4.Port4.Port_Discrete2_Count)SWPB(R95C.Read.IO_Metrics_1_to_4.Port4.Port_Discrete1_Totalizer,REVERSE,R95C.Read.IO_Metrics_1_to_4.Port4.Port_Discrete1_Totalizer)SWPB(R95C.Read.IO_Metrics_1_to_4.Port4.Port_Discrete1_Events_Per_Minute,REVERSE,R95C.Read.IO_Metrics_1_to_4.Port4.Port_Discrete1_Events_Per_Minute)SWPB(R95C.Read.IO_Metrics_1_to_4.Port4.Port_Discrete1_Duration,REVERSE,R95C.Read.IO_Metrics_1_to_4.Port4.Port_Discrete1_Duration)SWPB(R95C.Read.IO_Metrics_1_to_4.Port4.Port_Discrete1_Count,REVERSE,R95C.Read.IO_Metrics_1_to_4.Port4.Port_Discrete1_Count)SWPB(R95C.Read.IO_Metrics_1_to_4.Port3.Port_Discrete2_Totalizer,REVERSE,R95C.Read.IO_Metrics_1_to_4.Port3.Port_Discrete2_Totalizer)SWPB(R95C.Read.IO_Metrics_1_to_4.Port3.Port_Discrete2_Events_Per_Minute,REVERSE,R95C.Read.IO_Metrics_1_to_4.Port3.Port_Discrete2_Events_Per_Minute)SWPB(R95C.Read.IO_Metrics_1_to_4.Port3.Port_Discrete2_Duration,REVERSE,R95C.Read.IO_Metrics_1_to_4.Port3.Port_Discrete2_Duration)SWPB(R95C.Read.IO_Metrics_1_to_4.Port3.Port_Discrete2_Count,REVERSE,R95C.Read.IO_Metrics_1_to_4.Port3.Port_Discrete2_Count)SWPB(R95C.Read.IO_Metrics_1_to_4.Port3.Port_Discrete1_Totalizer,REVERSE,R95C.Read.IO_Metrics_1_to_4.Port3.Port_Discrete1_Totalizer)SWPB(R95C.Read.IO_Metrics_1_to_4.Port3.Port_Discrete1_Events_Per_Minute,REVERSE,R95C.Read.IO_Metrics_1_to_4.Port3.Port_Discrete1_Events_Per_Minute)SWPB(R95C.Read.IO_Metrics_1_to_4.Port3.Port_Discrete1_Duration,REVERSE,R95C.Read.IO_Metrics_1_to_4.Port3.Port_Discrete1_Duration)SWPB(R95C.Read.IO_Metrics_1_to_4.Port3.Port_Discrete1_Count,REVERSE,R95C.Read.IO_Metrics_1_to_4.Port3.Port_Discrete1_Count)SWPB(R95C.Read.IO_Metrics_1_to_4.Port2.Port_Discrete2_Totalizer,REVERSE,R95C.Read.IO_Metrics_1_to_4.Port2.Port_Discrete2_Totalizer)SWPB(R95C.Read.IO_Metrics_1_to_4.Port2.Port_Discrete2_Events_Per_Minute,REVERSE,R95C.Read.IO_Metrics_1_to_4.Port2.Port_Discrete2_Events_Per_Minute)SWPB(R95C.Read.IO_Metrics_1_to_4.Port2.Port_Discrete2_Duration,REVERSE,R95C.Read.IO_Metrics_1_to_4.Port2.Port_Discrete2_Duration)SWPB(R95C.Read.IO_Metrics_1_to_4.Port2.Port_Discrete2_Count,REVERSE,R95C.Read.IO_Metrics_1_to_4.Port2.Port_Discrete2_Count)SWPB(R95C.Read.IO_Metrics_1_to_4.Port2.Port_Discrete1_Totalizer,REVERSE,R95C.Read.IO_Metrics_1_to_4.Port2.Port_Discrete1_Totalizer)SWPB(R95C.Read.IO_Metrics_1_to_4.Port2.Port_Discrete1_Events_Per_Minute,REVERSE,R95C.Read.IO_Metrics_1_to_4.Port2.Port_Discrete1_Events_Per_Minute)SWPB(R95C.Read.IO_Metrics_1_to_4.Port2.Port_Discrete1_Duration,REVERSE,R95C.Read.IO_Metrics_1_to_4.Port2.Port_Discrete1_Duration)SWPB(R95C.Read.IO_Metrics_1_to_4.Port2.Port_Discrete1_Count,REVERSE,R95C.Read.IO_Metrics_1_to_4.Port2.Port_Discrete1_Count)SWPB(R95C.Read.IO_Metrics_1_to_4.Port1.Port_Discrete2_Totalizer,REVERSE,R95C.Read.IO_Metrics_1_to_4.Port1.Port_Discrete2_Totalizer)SWPB(R95C.Read.IO_Metrics_1_to_4.Port1.Port_Discrete2_Events_Per_Minute,REVERSE,R95C.Read.IO_Metrics_1_to_4.Port1.Port_Discrete2_Events_Per_Minute)SWPB(R95C.Read.IO_Metrics_1_to_4.Port1.Port_Discrete2_Duration,REVERSE,R95C.Read.IO_Metrics_1_to_4.Port1.Port_Discrete2_Duration)SWPB(R95C.Read.IO_Metrics_1_to_4.Port1.Port_Discrete2_Count,REVERSE,R95C.Read.IO_Metrics_1_to_4.Port1.Port_Discrete2_Count)SWPB(R95C.Read.IO_Metrics_1_to_4.Port1.Port_Discrete1_Totalizer,REVERSE,R95C.Read.IO_Metrics_1_to_4.Port1.Port_Discrete1_Totalizer)SWPB(R95C.Read.IO_Metrics_1_to_4.Port1.Port_Discrete1_Events_Per_Minute,REVERSE,R95C.Read.IO_Metrics_1_to_4.Port1.Port_Discrete1_Events_Per_Minute)SWPB(R95C.Read.IO_Metrics_1_to_4.Port1.Port_Discrete1_Duration,REVERSE,R95C.Read.IO_Metrics_1_to_4.Port1.Port_Discrete1_Duration)SWPB(R95C.Read.IO_Metrics_1_to_4.Port1.Port_Discrete1_Count,REVERSE,R95C.Read.IO_Metrics_1_to_4.Port1.Port_Discrete1_Count)OTU(Port_Data.Port_Read.[Port])OTL(Local_Control.6);
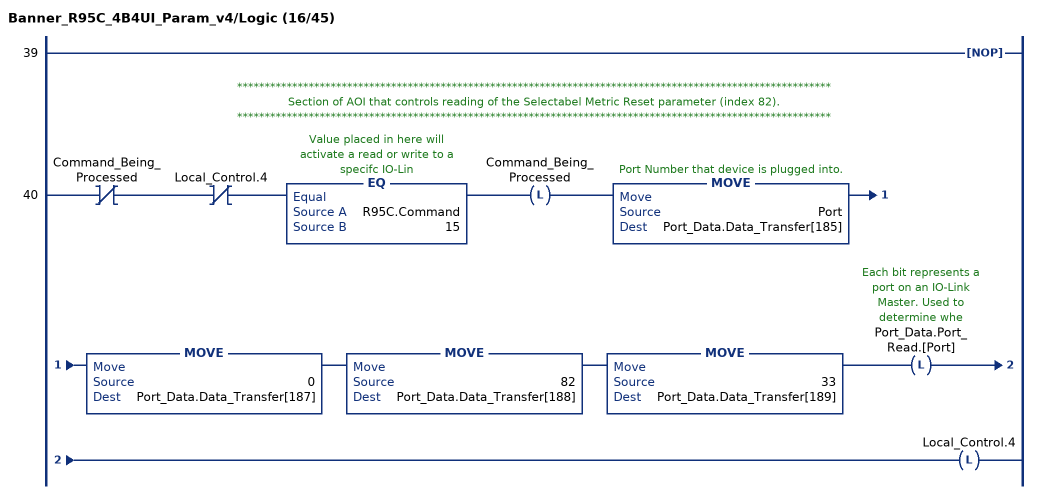
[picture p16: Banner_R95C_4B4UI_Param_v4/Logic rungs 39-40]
   39: NOP();
   // ************************************************************************************************************
   // Section of AOI that controls reading of the Selectabel Metric Reset parameter (index 82).
   // ************************************************************************************************************
   40: XIO(Command_Being_Processed)XIO(Local_Control.4)EQ(R95C.Command,15)OTL(Command_Being_Processed)MOVE(Port,Port_Data.Data_Transfer[185])MOVE(0,Port_Data.Data_Transfer[187])MOVE(82,Port_Data.Data_Transfer[188])MOVE(33,Port_Data.Data_Transfer[189])OTL(Port_Data.Port_Read.[Port])OTL(Local_Control.4);
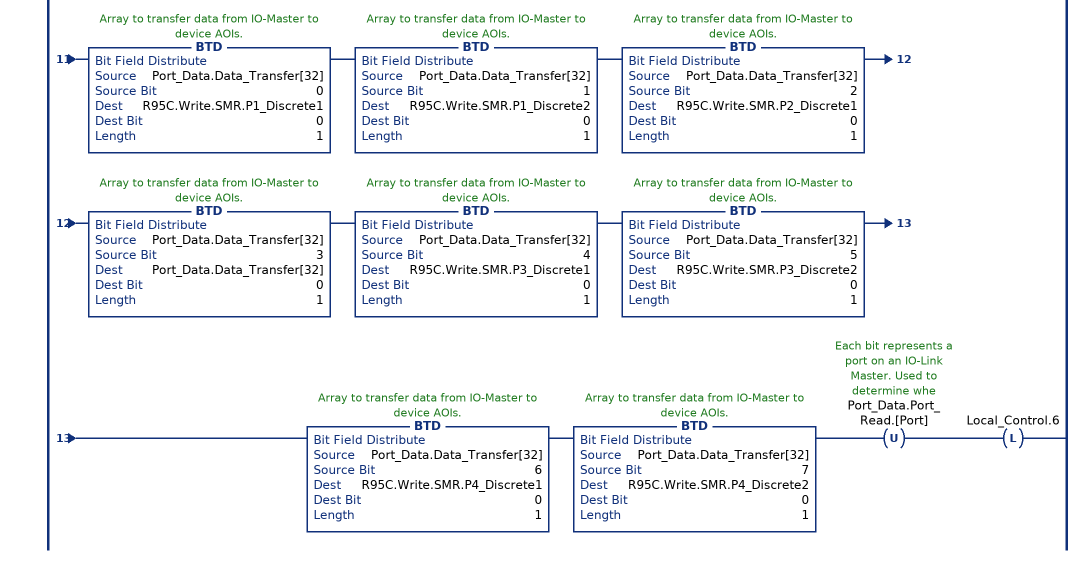
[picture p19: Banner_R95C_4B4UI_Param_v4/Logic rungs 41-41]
   41: XIC(Local_Control.5)XIO(Local_Control.6)EQ(R95C.Command,15)BTD(Port_Data.Data_Transfer[0],0,R95C.Write.SMR.P4_D2_Reset_Count,24,8)BTD(Port_Data.Data_Transfer[1],0,R95C.Write.SMR.P4_D2_Reset_Count,16,8)BTD(Port_Data.Data_Transfer[2],0,R95C.Write.SMR.P4_D2_Reset_Count,8,8)BTD(Port_Data.Data_Transfer[3],0,R95C.Write.SMR.P4_D2_Reset_Count,0,8)BTD(Port_Data.Data_Transfer[4],0,R95C.Write.SMR.P4_D1_Reset_Count,24,8)BTD(Port_Data.Data_Transfer[5],0,R95C.Write.SMR.P4_D1_Reset_Count,16,8)BTD(Port_Data.Data_Transfer[6],0,R95C.Write.SMR.P4_D1_Reset_Count,8,8)BTD(Port_Data.Data_Transfer[7],0,R95C.Write.SMR.P4_D1_Reset_Count,0,8)BTD(Port_Data.Data_Transfer[8],0,R95C.Write.SMR.P3_D2_Reset_Count,24,8)BTD(Port_Data.Data_Transfer[9],0,R95C.Write.SMR.P3_D2_Reset_Count,16,8)BTD(Port_Data.Data_Transfer[10],0,R95C.Write.SMR.P3_D2_Reset_Count,8,8)BTD(Port_Data.Data_Transfer[11],0,R95C.Write.SMR.P3_D2_Reset_Count,0,8)BTD(Port_Data.Data_Transfer[12],0,R95C.Write.SMR.P3_D1_Reset_Count,24,8)BTD(Port_Data.Data_Transfer[13],0,R95C.Write.SMR.P3_D1_Reset_Count,16,8)BTD(Port_Data.Data_Transfer[14],0,R95C.Write.SMR.P3_D1_Reset_Count,8,8)BTD(Port_Data.Data_Transfer[15],0,R95C.Write.SMR.P3_D1_Reset_Count,0,8)BTD(Port_Data.Data_Transfer[16],0,R95C.Write.SMR.P2_D2_Reset_Count,24,8)BTD(Port_Data.Data_Transfer[17],0,R95C.Write.SMR.P2_D2_Reset_Count,16,8)BTD(Port_Data.Data_Transfer[18],0,R95C.Write.SMR.P2_D2_Reset_Count,8,8)BTD(Port_Data.Data_Transfer[19],0,R95C.Write.SMR.P2_D2_Reset_Count,0,8)BTD(Port_Data.Data_Transfer[20],0,R95C.Write.SMR.P2_D1_Reset_Count,24,8)BTD(Port_Data.Data_Transfer[21],0,R95C.Write.SMR.P2_D1_Reset_Count,16,8)BTD(Port_Data.Data_Transfer[22],0,R95C.Write.SMR.P2_D1_Reset_Count,8,8)BTD(Port_Data.Data_Transfer[23],0,R95C.Write.SMR.P2_D1_Reset_Count,0,8)BTD(Port_Data.Data_Transfer[24],0,R95C.Write.SMR.P1_D2_Reset_Count,24,8)BTD(Port_Data.Data_Transfer[25],0,R95C.Write.SMR.P1_D2_Reset_Count,16,8)BTD(Port_Data.Data_Transfer[26],0,R95C.Write.SMR.P1_D2_Reset_Count,8,8)BTD(Port_Data.Data_Transfer[27],0,R95C.Write.SMR.P1_D2_Reset_Count,0,8)BTD(Port_Data.Data_Transfer[28],0,R95C.Write.SMR.P1_D1_Reset_Count,24,8)BTD(Port_Data.Data_Transfer[29],0,R95C.Write.SMR.P1_D1_Reset_Count,16,8)BTD(Port_Data.Data_Transfer[30],0,R95C.Write.SMR.P1_D1_Reset_Count,8,8)BTD(Port_Data.Data_Transfer[31],0,R95C.Write.SMR.P1_D1_Reset_Count,0,8)BTD(Port_Data.Data_Transfer[32],0,R95C.Write.SMR.P1_Discrete1,0,1)BTD(Port_Data.Data_Transfer[32],1,R95C.Write.SMR.P1_Discrete2,0,1)BTD(Port_Data.Data_Transfer[32],2,R95C.Write.SMR.P2_Discrete1,0,1)BTD(Port_Data.Data_Transfer[32],3,Port_Data.Data_Transfer[32],0,1)BTD(Port_Data.Data_Transfer[32],4,R95C.Write.SMR.P3_Discrete1,0,1)BTD(Port_Data.Data_Transfer[32],5,R95C.Write.SMR.P3_Discrete2,0,1)BTD(Port_Data.Data_Transfer[32],6,R95C.Write.SMR.P4_Discrete1,0,1)BTD(Port_Data.Data_Transfer[32],7,R95C.Write.SMR.P4_Discrete2,0,1)OTU(Port_Data.Port_Read.[Port])OTL(Local_Control.6);
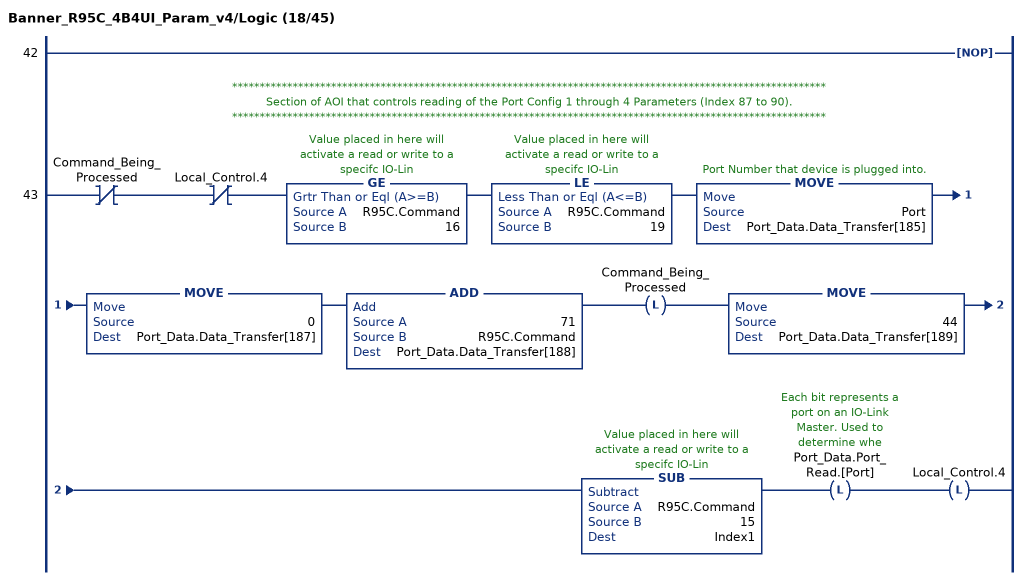
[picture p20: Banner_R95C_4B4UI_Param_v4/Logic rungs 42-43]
   42: NOP();
   // ************************************************************************************************************
   // Section of AOI that controls reading of the Port Config 1 through 4 Parameters (Index 87 to 90).
   // ************************************************************************************************************
   43: XIO(Command_Being_Processed)XIO(Local_Control.4)GE(R95C.Command,16)LE(R95C.Command,19)MOVE(Port,Port_Data.Data_Transfer[185])MOVE(0,Port_Data.Data_Transfer[187])ADD(71,R95C.Command,Port_Data.Data_Transfer[188])OTL(Command_Being_Processed)MOVE(44,Port_Data.Data_Transfer[189])SUB(R95C.Command,15,Index1)OTL(Port_Data.Port_Read.[Port])OTL(Local_Control.4);
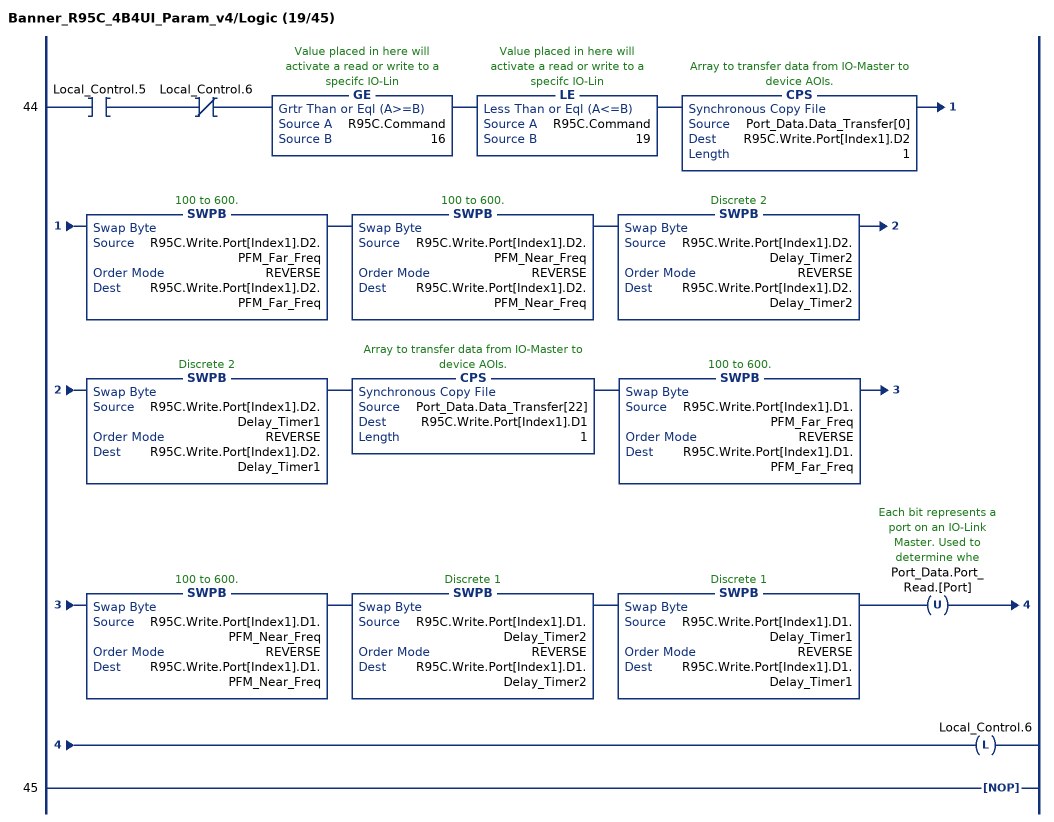
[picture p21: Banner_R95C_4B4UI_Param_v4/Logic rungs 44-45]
   44: XIC(Local_Control.5)XIO(Local_Control.6)GE(R95C.Command,16)LE(R95C.Command,19)CPS(Port_Data.Data_Transfer[0],R95C.Write.Port[Index1].D2,1)SWPB(R95C.Write.Port[Index1].D2.PFM_Far_Freq,REVERSE,R95C.Write.Port[Index1].D2.PFM_Far_Freq)SWPB(R95C.Write.Port[Index1].D2.PFM_Near_Freq,REVERSE,R95C.Write.Port[Index1].D2.PFM_Near_Freq)SWPB(R95C.Write.Port[Index1].D2.Delay_Timer2,REVERSE,R95C.Write.Port[Index1].D2.Delay_Timer2)SWPB(R95C.Write.Port[Index1].D2.Delay_Timer1,REVERSE,R95C.Write.Port[Index1].D2.Delay_Timer1)CPS(Port_Data.Data_Transfer[22],R95C.Write.Port[Index1].D1,1)SWPB(R95C.Write.Port[Index1].D1.PFM_Far_Freq,REVERSE,R95C.Write.Port[Index1].D1.PFM_Far_Freq)SWPB(R95C.Write.Port[Index1].D1.PFM_Near_Freq,REVERSE,R95C.Write.Port[Index1].D1.PFM_Near_Freq)SWPB(R95C.Write.Port[Index1].D1.Delay_Timer2,REVERSE,R95C.Write.Port[Index1].D1.Delay_Timer2)SWPB(R95C.Write.Port[Index1].D1.Delay_Timer1,REVERSE,R95C.Write.Port[Index1].D1.Delay_Timer1)OTU(Port_Data.Port_Read.[Port])OTL(Local_Control.6);
   45: NOP();
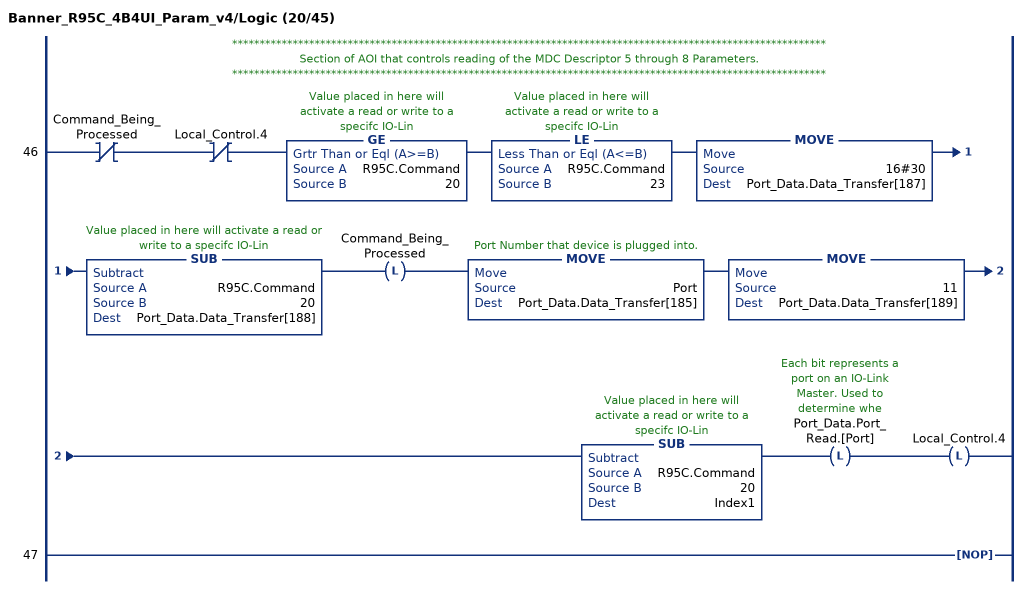
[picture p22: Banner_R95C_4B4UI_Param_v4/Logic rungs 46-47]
   // ************************************************************************************************************
   // Section of AOI that controls reading of the MDC Descriptor 5 through 8 Parameters.
   // ************************************************************************************************************
   46: XIO(Command_Being_Processed)XIO(Local_Control.4)GE(R95C.Command,20)LE(R95C.Command,23)MOVE(16#30,Port_Data.Data_Transfer[187])SUB(R95C.Command,20,Port_Data.Data_Transfer[188])OTL(Command_Being_Processed)MOVE(Port,Port_Data.Data_Transfer[185])MOVE(11,Port_Data.Data_Transfer[189])SUB(R95C.Command,20,Index1)OTL(Port_Data.Port_Read.[Port])OTL(Local_Control.4);
   47: NOP();
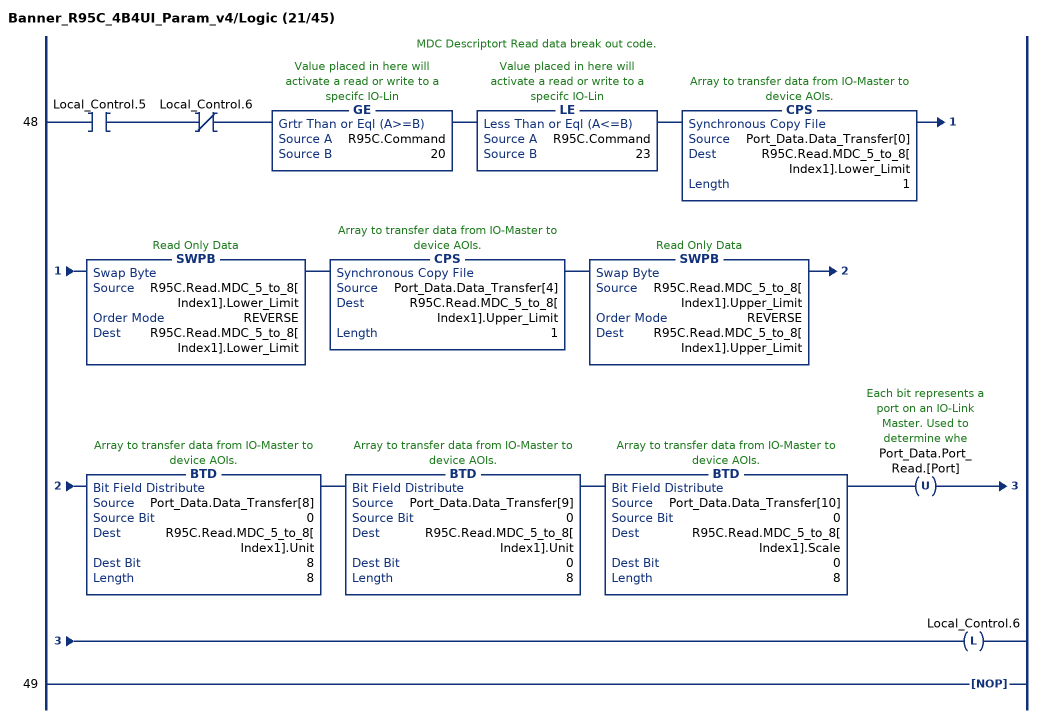
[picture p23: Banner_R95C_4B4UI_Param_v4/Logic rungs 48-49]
   // MDC Descriptort Read data break out code.
   48: XIC(Local_Control.5)XIO(Local_Control.6)GE(R95C.Command,20)LE(R95C.Command,23)CPS(Port_Data.Data_Transfer[0],R95C.Read.MDC_5_to_8[Index1].Lower_Limit,1)SWPB(R95C.Read.MDC_5_to_8[Index1].Lower_Limit,REVERSE,R95C.Read.MDC_5_to_8[Index1].Lower_Limit)CPS(Port_Data.Data_Transfer[4],R95C.Read.MDC_5_to_8[Index1].Upper_Limit,1)SWPB(R95C.Read.MDC_5_to_8[Index1].Upper_Limit,REVERSE,R95C.Read.MDC_5_to_8[Index1].Upper_Limit)BTD(Port_Data.Data_Transfer[8],0,R95C.Read.MDC_5_to_8[Index1].Unit,8,8)BTD(Port_Data.Data_Transfer[9],0,R95C.Read.MDC_5_to_8[Index1].Unit,0,8)BTD(Port_Data.Data_Transfer[10],0,R95C.Read.MDC_5_to_8[Index1].Scale,0,8)OTU(Port_Data.Port_Read.[Port])OTL(Local_Control.6);
   49: NOP();
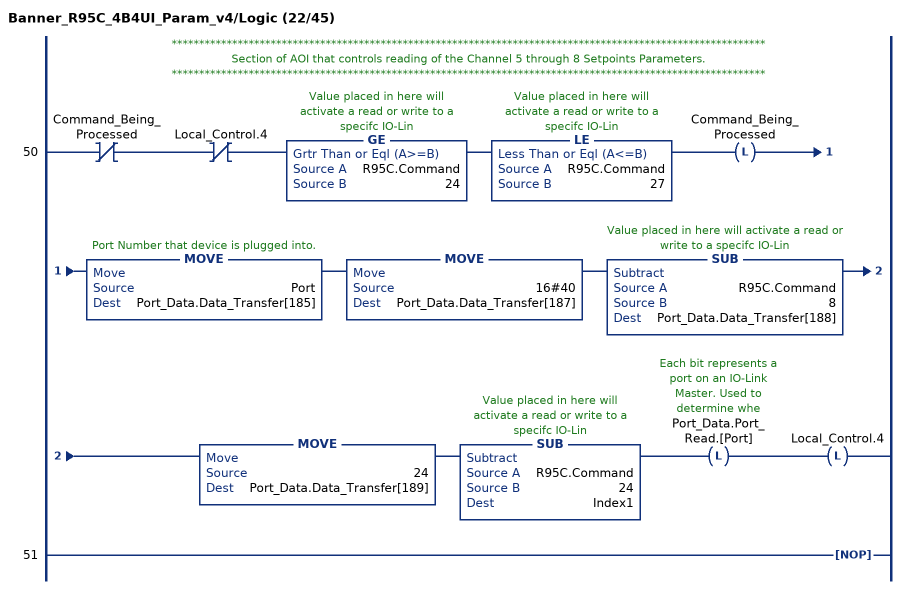
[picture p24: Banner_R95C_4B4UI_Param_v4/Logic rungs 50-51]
   // ************************************************************************************************************
   // Section of AOI that controls reading of the Channel 5 through 8 Setpoints Parameters.
   // ************************************************************************************************************
   50: XIO(Command_Being_Processed)XIO(Local_Control.4)GE(R95C.Command,24)LE(R95C.Command,27)OTL(Command_Being_Processed)MOVE(Port,Port_Data.Data_Transfer[185])MOVE(16#40,Port_Data.Data_Transfer[187])SUB(R95C.Command,8,Port_Data.Data_Transfer[188])MOVE(24,Port_Data.Data_Transfer[189])SUB(R95C.Command,24,Index1)OTL(Port_Data.Port_Read.[Port])OTL(Local_Control.4);
   51: NOP();
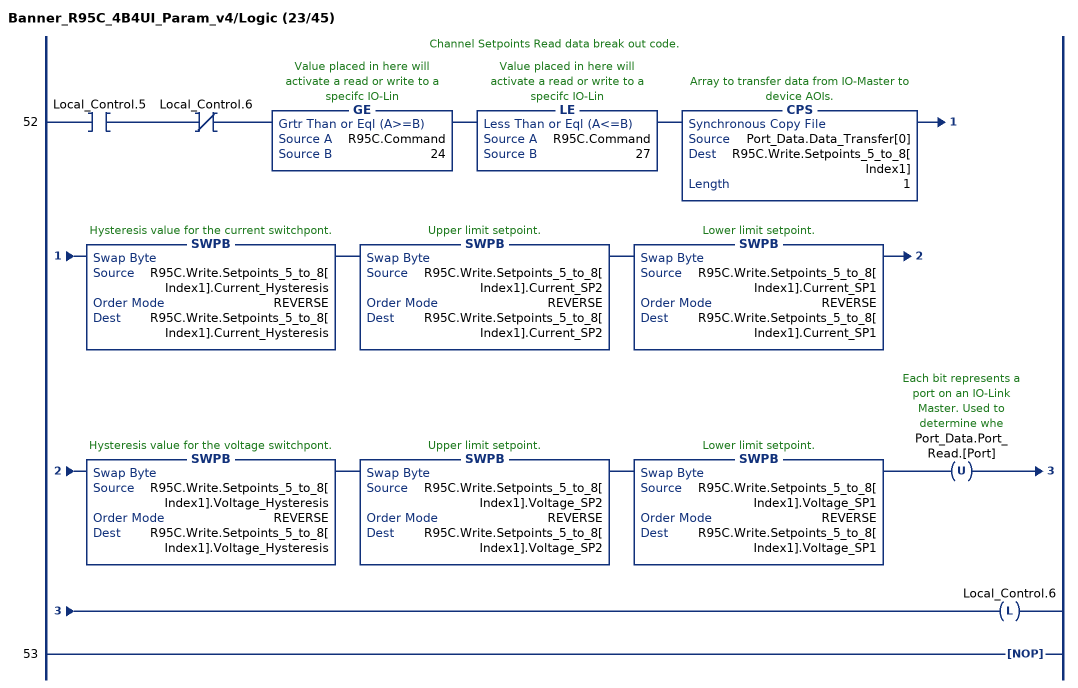
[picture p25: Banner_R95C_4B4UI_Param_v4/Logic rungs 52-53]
   // Channel Setpoints Read data break out code.
   52: XIC(Local_Control.5)XIO(Local_Control.6)GE(R95C.Command,24)LE(R95C.Command,27)CPS(Port_Data.Data_Transfer[0],R95C.Write.Setpoints_5_to_8[Index1],1)SWPB(R95C.Write.Setpoints_5_to_8[Index1].Current_Hysteresis,REVERSE,R95C.Write.Setpoints_5_to_8[Index1].Current_Hysteresis)SWPB(R95C.Write.Setpoints_5_to_8[Index1].Current_SP2,REVERSE,R95C.Write.Setpoints_5_to_8[Index1].Current_SP2)SWPB(R95C.Write.Setpoints_5_to_8[Index1].Current_SP1,REVERSE,R95C.Write.Setpoints_5_to_8[Index1].Current_SP1)SWPB(R95C.Write.Setpoints_5_to_8[Index1].Voltage_Hysteresis,REVERSE,R95C.Write.Setpoints_5_to_8[Index1].Voltage_Hysteresis)SWPB(R95C.Write.Setpoints_5_to_8[Index1].Voltage_SP2,REVERSE,R95C.Write.Setpoints_5_to_8[Index1].Voltage_SP2)SWPB(R95C.Write.Setpoints_5_to_8[Index1].Voltage_SP1,REVERSE,R95C.Write.Setpoints_5_to_8[Index1].Voltage_SP1)OTU(Port_Data.Port_Read.[Port])OTL(Local_Control.6);
   53: NOP();
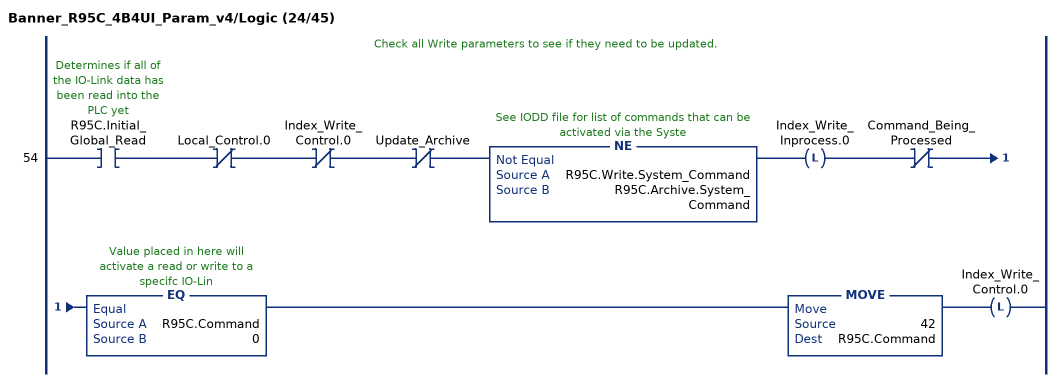
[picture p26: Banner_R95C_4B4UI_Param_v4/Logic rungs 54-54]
   // Check all Write parameters to see if they need to be updated.
   54: XIC(R95C.Initial_Global_Read)XIO(Local_Control.0)XIO(Index_Write_Control.0)XIO(Update_Archive)NE(R95C.Write.System_Command,R95C.Archive.System_Command)OTL(Index_Write_Inprocess.0)XIO(Command_Being_Processed)EQ(R95C.Command,0)MOVE(42,R95C.Command)OTL(Index_Write_Control.0);
